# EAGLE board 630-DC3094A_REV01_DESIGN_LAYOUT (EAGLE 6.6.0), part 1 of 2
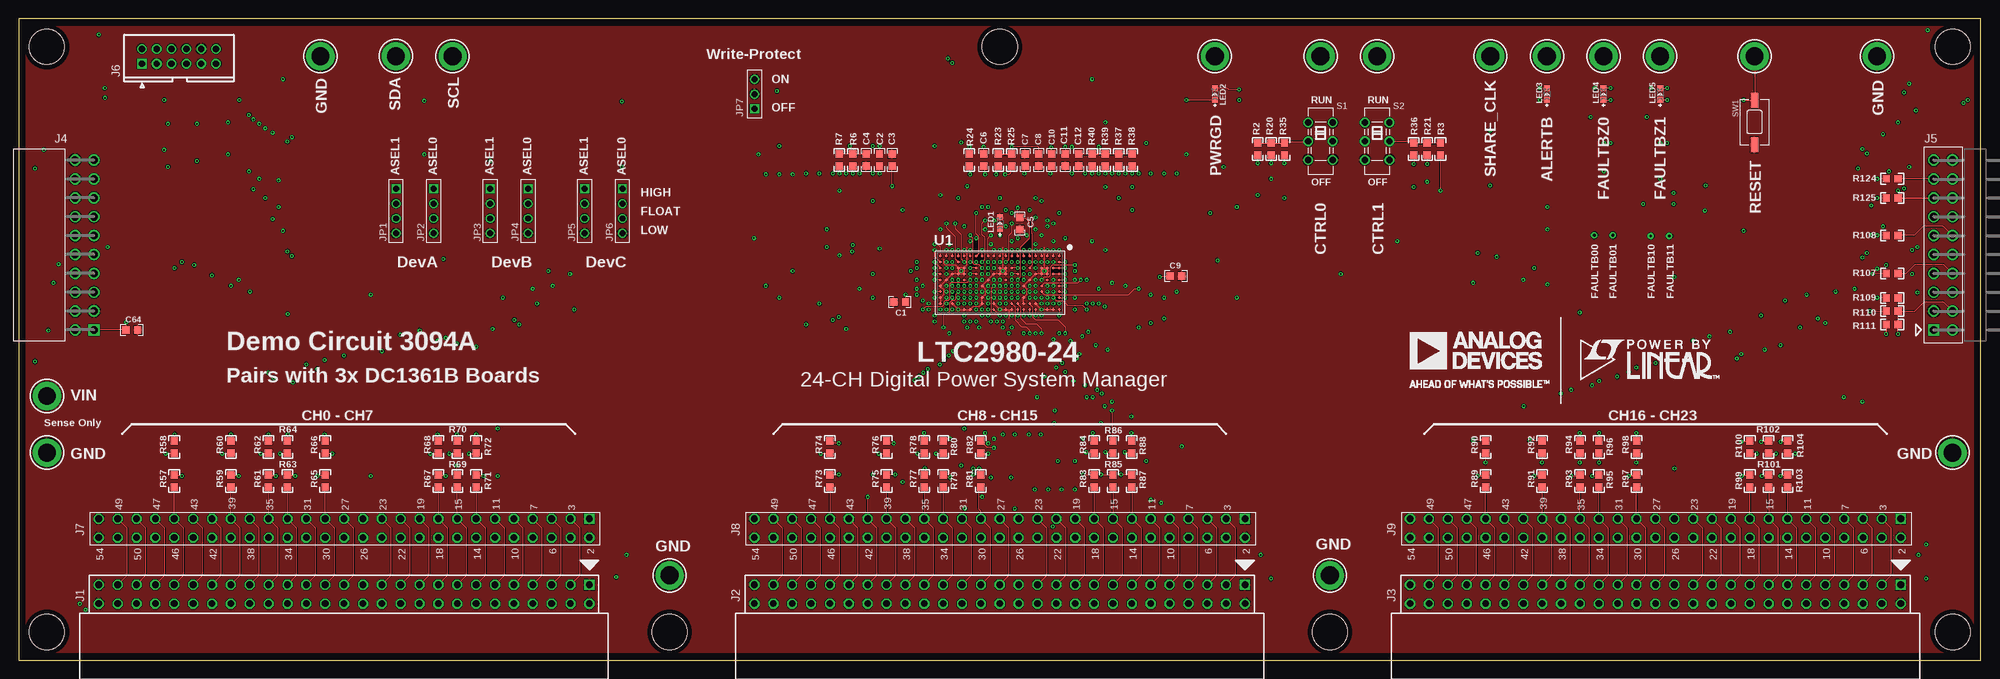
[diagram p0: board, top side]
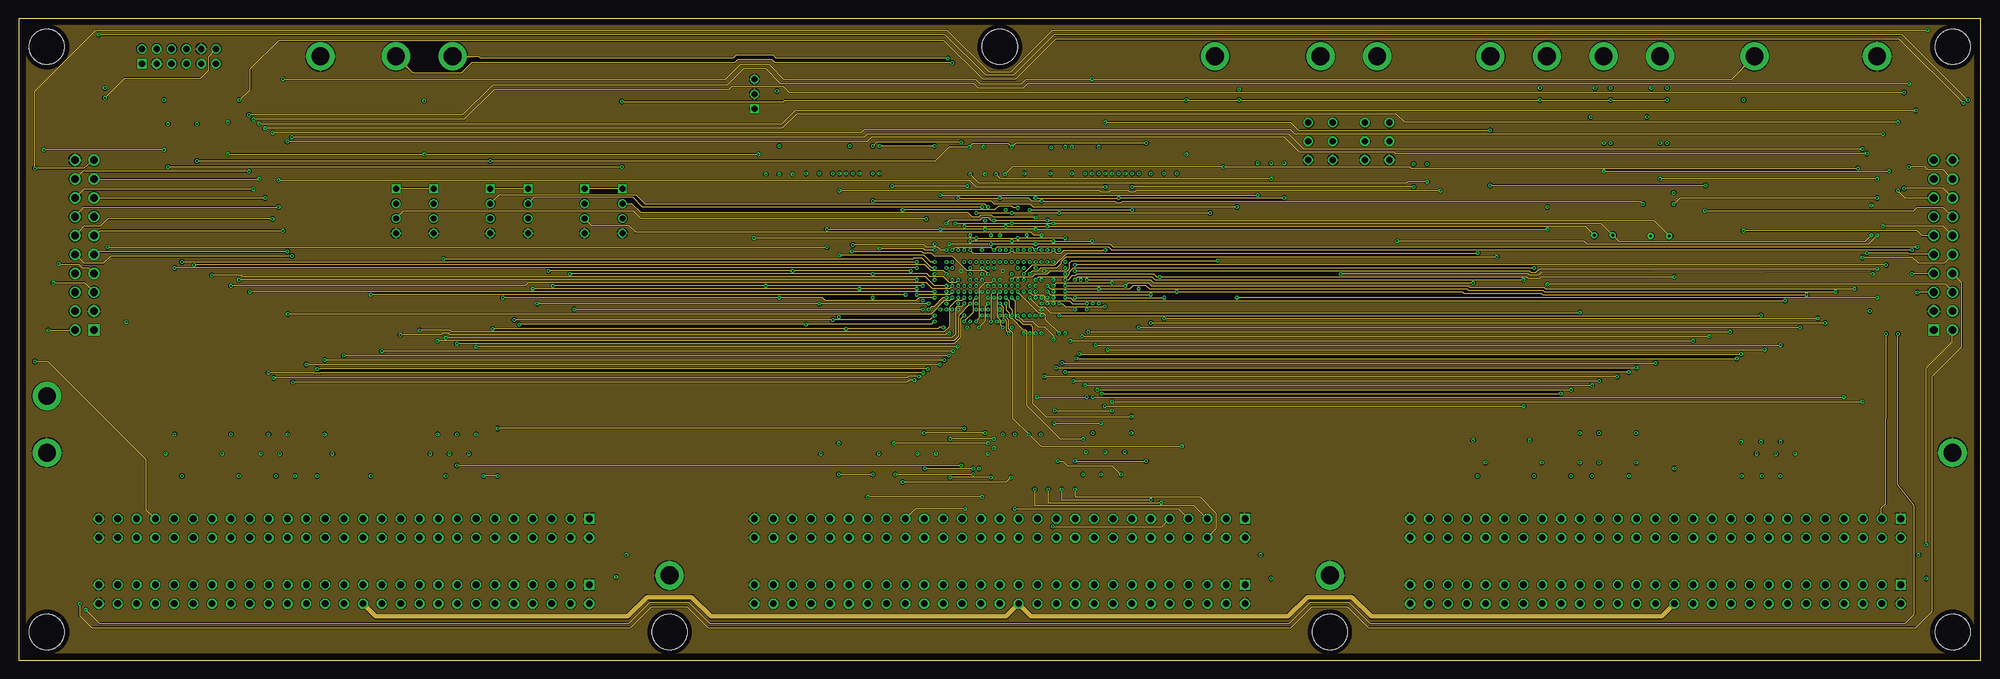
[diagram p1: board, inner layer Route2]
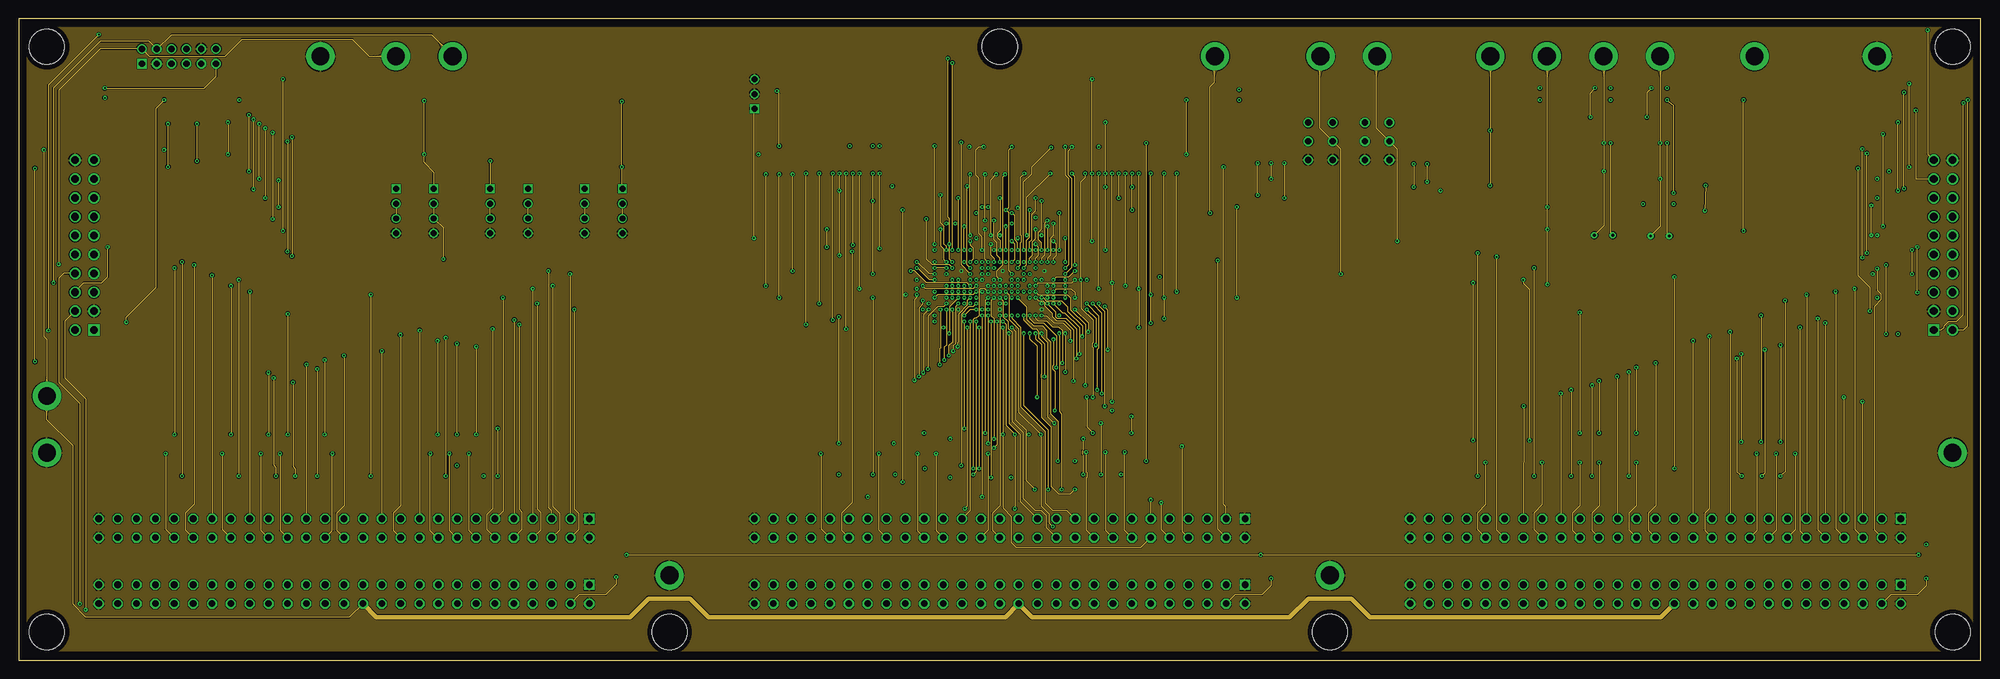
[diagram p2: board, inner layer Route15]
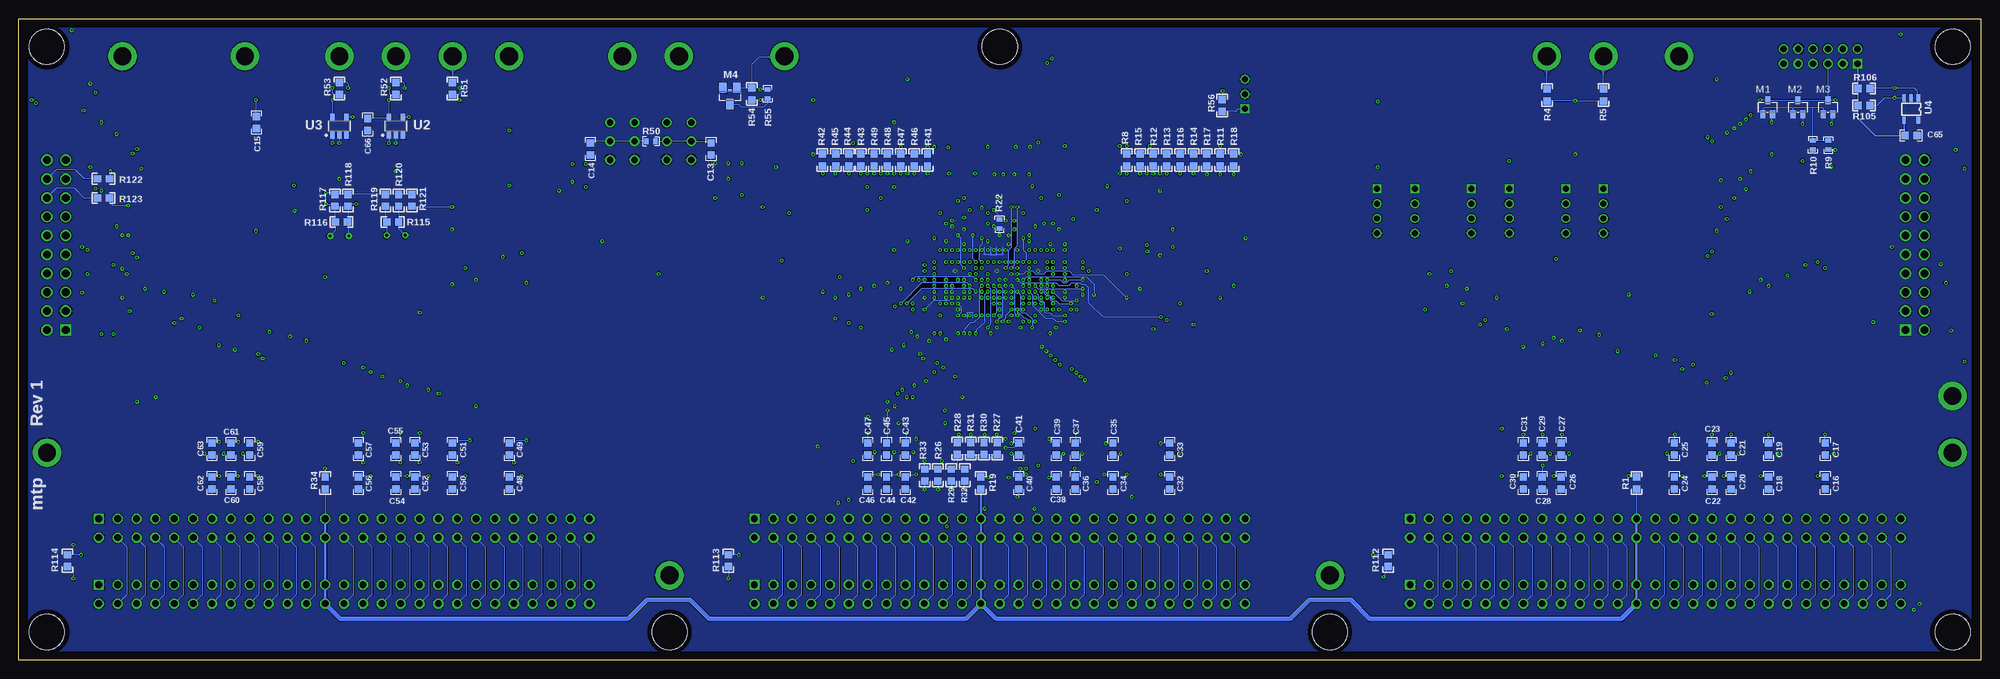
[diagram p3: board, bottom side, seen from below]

Size 264.16 x 86.36 mm. Coordinates in mm from the lower left corner, seen from the top.
Outline: 0,0 264.16,0 264.16,86.36 0,86.36 0,0
Copper layers (1*2+15*16): Top 0.035mm / dielectric 0.25mm / Route2 0.035mm / dielectric 0.9mm / Route15 0.035mm / dielectric 0.25mm / Bottom 0.035mm
Design rules "default *": minimum track width 0.1mm, minimum drill 0.2mm, track to track 0.1mm, track to pad 0.1mm, pad to pad 0.1mm, via to via 0.1mm, smd to smd 0mil, copper to edge 24mil, drill to drill 0.5mm, minimum pad ring 0.15mm, minimum via ring 0.15mm, stop-mask expansion 4mil, vias tented up to drill 10mil, thermal gap 0.15mm
Holes 4.75 mm at 3.81,3.81 3.81,82.55 260.35,82.55 260.35,3.81 87.63,3.81 176.53,3.81 132.08,82.55

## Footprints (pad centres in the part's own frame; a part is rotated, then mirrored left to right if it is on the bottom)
C0603_BOX = smd 1 x 1: 1 -0.8,0; 2 0.8,0
PINHEAD_2X27_RECEPTACLE = drill 0.9 square: 1 1.27,-33.02 | drill 0.9 octagon: 2 -1.27,-33.02; 3 1.27,-30.48; 4 -1.27,-30.48; 5 1.27,-27.94; 6 -1.27,-27.94; 7 1.27,-25.4; 8 -1.27,-25.4; 9 1.27,-22.86; 10 -1.27,-22.86; 11 1.27,-20.32; 12 -1.27,-20.32; 13 1.27,-17.78; 14 -1.27,-17.78; 15 1.27,-15.24; 16 -1.27,-15.24; 17 1.27,-12.7; 18 -1.27,-12.7; 19 1.27,-10.16; 20 -1.27,-10.16; 21 1.27,-7.62; 22 -1.27,-7.62; 23 1.27,-5.08; 24 -1.27,-5.08; 25 1.27,-2.54; 26 -1.27,-2.54; 27 1.27,0; 28 -1.27,0; 29 1.27,2.54; 30 -1.27,2.54; 31 1.27,5.08; 32 -1.27,5.08; 33 1.27,7.62; 34 -1.27,7.62; 35 1.27,10.16; 36 -1.27,10.16; 37 1.27,12.7; 38 -1.27,12.7; 39 1.27,15.24; 40 -1.27,15.24; 41 1.27,17.78; 42 -1.27,17.78; 43 1.27,20.32; 44 -1.27,20.32; 45 1.27,22.86; 46 -1.27,22.86; 47 1.27,25.4; 48 -1.27,25.4; 49 1.27,27.94; 50 -1.27,27.94; 51 1.27,30.48; 52 -1.27,30.48; 53 1.27,33.02; 54 -1.27,33.02
RECEPT_2X10_0.1INCH = drill 1.016 square: P$1 -1.27,11.43 | drill 1.016: P$2 1.27,11.43; P$3 -1.27,8.89; P$4 1.27,8.89; P$5 -1.27,6.35; P$6 1.27,6.35; P$7 -1.27,3.81; P$8 1.27,3.81; P$9 -1.27,1.27; P$10 1.27,1.27; P$11 -1.27,-1.27; P$12 1.27,-1.27; P$13 -1.27,-3.81; P$14 1.27,-3.81; P$15 -1.27,-6.35; P$16 1.27,-6.35; P$17 -1.27,-8.89; P$18 1.27,-8.89; P$19 -1.27,-11.43; P$20 1.27,-11.43
HEADER_2X10_0.1INCH = drill 1.016 square: P$1 1.27,11.43 | drill 1.016: P$2 -1.27,11.43; P$3 1.27,8.89; P$4 -1.27,8.89; P$5 1.27,6.35; P$6 -1.27,6.35; P$7 1.27,3.81; P$8 -1.27,3.81; P$9 1.27,1.27; P$10 -1.27,1.27; P$11 1.27,-1.27; P$12 -1.27,-1.27; P$13 1.27,-3.81; P$14 -1.27,-3.81; P$15 1.27,-6.35; P$16 -1.27,-6.35; P$17 1.27,-8.89; P$18 -1.27,-8.89; P$19 1.27,-11.43; P$20 -1.27,-11.43
CONN_DC1613 = drill 0.86 square: 1 -5,-1 | drill 0.86: 2 -5,1; 3 -3,-1; 4 -3,1; 5 -1,-1; 6 -1,1; 7 1,-1; 8 1,1; 9 3,-1; 10 3,1; 11 5,-1; 12 5,1
PINHEAD_2X27_RECEPTACLE_NO_SILK = drill 0.9 square: 1 1.27,-33.02 | drill 0.9 octagon: 2 -1.27,-33.02; 3 1.27,-30.48; 4 -1.27,-30.48; 5 1.27,-27.94; 6 -1.27,-27.94; 7 1.27,-25.4; 8 -1.27,-25.4; 9 1.27,-22.86; 10 -1.27,-22.86; 11 1.27,-20.32; 12 -1.27,-20.32; 13 1.27,-17.78; 14 -1.27,-17.78; 15 1.27,-15.24; 16 -1.27,-15.24; 17 1.27,-12.7; 18 -1.27,-12.7; 19 1.27,-10.16; 20 -1.27,-10.16; 21 1.27,-7.62; 22 -1.27,-7.62; 23 1.27,-5.08; 24 -1.27,-5.08; 25 1.27,-2.54; 26 -1.27,-2.54; 27 1.27,0; 28 -1.27,0; 29 1.27,2.54; 30 -1.27,2.54; 31 1.27,5.08; 32 -1.27,5.08; 33 1.27,7.62; 34 -1.27,7.62; 35 1.27,10.16; 36 -1.27,10.16; 37 1.27,12.7; 38 -1.27,12.7; 39 1.27,15.24; 40 -1.27,15.24; 41 1.27,17.78; 42 -1.27,17.78; 43 1.27,20.32; 44 -1.27,20.32; 45 1.27,22.86; 46 -1.27,22.86; 47 1.27,25.4; 48 -1.27,25.4; 49 1.27,27.94; 50 -1.27,27.94; 51 1.27,30.48; 52 -1.27,30.48; 53 1.27,33.02; 54 -1.27,33.02
1X04-2MM = drill 0.8 square: 1 -3,0 | drill 0.8: 2 -1,0; 3 1,0; 4 3,0
1X03-2MM = drill 0.8 square: 1 -2,0 | drill 0.8: 2 0,0; 3 2,0
CHIPLED_0603 = smd 0.8 x 0.8: N 0,0.78; P 0,-0.78
SOT323@1 = smd 0.7 x 1.1: 1 -0.65,-0.95; 2 0.65,-0.95; 3 0,0.95
SOT23 = smd 1 x 1.4: 1 -0.95,-1.1; 2 0.95,-1.1; 3 0,1.1
R0603_BOX = smd 1 x 1: 1 -0.8,0; 2 0.8,0
R0402_BOX = smd 0.6 x 0.8: 1 -0.6,0; 2 0.6,0
JS202011CQN = drill 0.86: 1 -2.5,1.65; 2 0,1.65; 3 2.5,1.65; 4 -2.5,-1.65; 5 0,-1.65; 6 2.5,-1.65
SWITCH_PTS635 = smd 2 x 1: SW1 -3,0; SW2 3,0
TURRET_LARGE_2501 = drill 2.388 pad 3.81: TP 0,0
VIA = drill 0.381 pad 0.864: 1 0,0
BGA210 = smd 0.4 x 0.4: A1 -8,-3.6; A2 -8,-2.8; A3 -8,-2; A4 -8,-1.2; A5 -8,-0.4; A6 -8,0.4; A7 -8,1.2; A8 -8,2; A9 -8,2.8; A10 -8,3.6; B1 -7.2,-3.6; B2 -7.2,-2.8; B3 -7.2,-2; B4 -7.2,-1.2; B5 -7.2,-0.4; B6 -7.2,0.4; B7 -7.2,1.2; B8 -7.2,2; B9 -7.2,2.8; B10 -7.2,3.6; C1 -6.4,-3.6; C2 -6.4,-2.8; C3 -6.4,-2; C4 -6.4,-1.2; C5 -6.4,-0.4; C6 -6.4,0.4; C7 -6.4,1.2; C8 -6.4,2; C9 -6.4,2.8; C10 -6.4,3.6; D1 -5.6,-3.6; D2 -5.6,-2.8; D3 -5.6,-2; D4 -5.6,-1.2; D5 -5.6,-0.4; D6 -5.6,0.4; D7 -5.6,1.2; D8 -5.6,2; D9 -5.6,2.8; D10 -5.6,3.6; E1 -4.8,-3.6; E2 -4.8,-2.8; E3 -4.8,-2; E4 -4.8,-1.2; E5 -4.8,-0.4; E6 -4.8,0.4; E7 -4.8,1.2; E8 -4.8,2; E9 -4.8,2.8; E10 -4.8,3.6; F1 -4,-3.6; F2 -4,-2.8; F3 -4,-2; F4 -4,-1.2; F5 -4,-0.4; F6 -4,0.4; F7 -4,1.2; F8 -4,2; F9 -4,2.8; F10 -4,3.6; G1 -3.2,-3.6; G2 -3.2,-2.8; G3 -3.2,-2; G4 -3.2,-1.2; G5 -3.2,-0.4; G6 -3.2,0.4; G7 -3.2,1.2; G8 -3.2,2; G9 -3.2,2.8; G10 -3.2,3.6; H1 -2.4,-3.6; H2 -2.4,-2.8; H3 -2.4,-2; H4 -2.4,-1.2; H5 -2.4,-0.4; H6 -2.4,0.4; H7 -2.4,1.2; H8 -2.4,2; H9 -2.4,2.8; H10 -2.4,3.6; J1 -1.6,-3.6; J2 -1.6,-2.8; J3 -1.6,-2; J4 -1.6,-1.2; J5 -1.6,-0.4; J6 -1.6,0.4; J7 -1.6,1.2; J8 -1.6,2; J9 -1.6,2.8; J10 -1.6,3.6; K1 -0.8,-3.6; K2 -0.8,-2.8; K3 -0.8,-2; K4 -0.8,-1.2; K5 -0.8,-0.4; K6 -0.8,0.4; K7 -0.8,1.2; K8 -0.8,2; K9 -0.8,2.8; K10 -0.8,3.6; L1 0,-3.6; L2 0,-2.8; L3 0,-2; L4 0,-1.2; L5 0,-0.4; L6 0,0.4; L7 0,1.2; L8 0,2; L9 0,2.8; L10 0,3.6; M1 0.8,-3.6; M2 0.8,-2.8; M3 0.8,-2; M4 0.8,-1.2; M5 0.8,-0.4; M6 0.8,0.4; M7 0.8,1.2; M8 0.8,2; M9 0.8,2.8; M10 0.8,3.6; N1 1.6,-3.6; N2 1.6,-2.8; N3 1.6,-2; N4 1.6,-1.2; N5 1.6,-0.4; N6 1.6,0.4; N7 1.6,1.2; N8 1.6,2; N9 1.6,2.8; N10 1.6,3.6; P1 2.4,-3.6; P2 2.4,-2.8; P3 2.4,-2; P4 2.4,-1.2; P5 2.4,-0.4; P6 2.4,0.4; P7 2.4,1.2; P8 2.4,2; P9 2.4,2.8; P10 2.4,3.6; R1 3.2,-3.6; R2 3.2,-2.8; R3 3.2,-2; R4 3.2,-1.2; R5 3.2,-0.4; R6 3.2,0.4; R7 3.2,1.2; R8 3.2,2; R9 3.2,2.8; R10 3.2,3.6; T1 4,-3.6; T2 4,-2.8; T3 4,-2; T4 4,-1.2; T5 4,-0.4; T6 4,0.4; T7 4,1.2; T8 4,2; T9 4,2.8; T10 4,3.6; U1 4.8,-3.6; U2 4.8,-2.8; U3 4.8,-2; U4 4.8,-1.2; U5 4.8,-0.4; U6 4.8,0.4; U7 4.8,1.2; U8 4.8,2; U9 4.8,2.8; U10 4.8,3.6; W1 5.6,-3.6; W2 5.6,-2.8; W3 5.6,-2; W4 5.6,-1.2; W5 5.6,-0.4; W6 5.6,0.4; W7 5.6,1.2; W8 5.6,2; W9 5.6,2.8; W10 5.6,3.6; X1 6.4,-3.6; X2 6.4,-2.8; X3 6.4,-2; X4 6.4,-1.2; X5 6.4,-0.4; X6 6.4,0.4; X7 6.4,1.2; X8 6.4,2; X9 6.4,2.8; X10 6.4,3.6; Y1 7.2,-3.6; Y2 7.2,-2.8; Y3 7.2,-2; Y4 7.2,-1.2; Y5 7.2,-0.4; Y6 7.2,0.4; Y7 7.2,1.2; Y8 7.2,2; Y9 7.2,2.8; Y10 7.2,3.6; Z1 8,-3.6; Z2 8,-2.8; Z3 8,-2; Z4 8,-1.2; Z5 8,-0.4; Z6 8,0.4; Z7 8,1.2; Z8 8,2; Z9 8,2.8; Z10 8,3.6
SOT23-5 = smd 0.6 x 1: 1 -0.95,-1.2; 2 0,-1.2; 3 0.95,-1.2; 4 0.95,1.2; 5 -0.95,1.2
SOT-23-5 = smd 1 x 0.5: 1 -1.491,0.95; 2 -1.491,0; 3 -1.491,-0.95; 4 1.491,-0.95; 5 1.491,0.95

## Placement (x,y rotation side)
C1  0.1uF  [C0603_BOX]  118.6,48.2 180 top
C2  0.1uF  [C0603_BOX]  115.9,67.31 90 top
C3  0.1uF  [C0603_BOX]  117.6,67.31 90 top
C4  0.1uF  [C0603_BOX]  114.1,67.31 270 top
C5  0.1uF  [C0603_BOX]  134.8,58.8 270 top
C6  0.1uF  [C0603_BOX]  129.9,67.31 90 top
C7  0.1uF  [C0603_BOX]  135.5,67.31 90 top
C8  0.1uF  [C0603_BOX]  137.3,67.31 270 top
C9  0.1uF  [C0603_BOX]  155.8,51.7 0 top
C10  0.1uF  [C0603_BOX]  139.09,67.31 90 top
C11  0.1uF  [C0603_BOX]  140.9,67.31 270 top
C12  0.1uF  [C0603_BOX]  142.7,67.31 270 top
C13  1uF  [C0603_BOX]  170.94,68.8 270 bottom
C14  1uF  [C0603_BOX]  187.2,68.8 270 bottom
C15  10n  [C0603_BOX]  232.16,72.39 90 bottom
C16  100n  [C0603_BOX]  20.95,23.88 270 bottom
C17  100n  [C0603_BOX]  20.95,28.45 270 bottom
C18  100n  [C0603_BOX]  28.57,23.88 270 bottom
C19  100n  [C0603_BOX]  28.57,28.45 270 bottom
C20  100n  [C0603_BOX]  33.66,23.88 270 bottom
C21  100n  [C0603_BOX]  33.66,28.45 270 bottom
C22  100n  [C0603_BOX]  36.2,23.88 270 bottom
C23  100n  [C0603_BOX]  36.2,28.45 270 bottom
C24  100n  [C0603_BOX]  41.27,23.88 270 bottom
C25  100n  [C0603_BOX]  41.27,28.45 270 bottom
C26  100n  [C0603_BOX]  56.52,23.88 270 bottom
C27  100n  [C0603_BOX]  56.52,28.45 270 bottom
C28  100n  [C0603_BOX]  59.05,23.88 270 bottom
C29  100n  [C0603_BOX]  59.05,28.45 270 bottom
C30  100n  [C0603_BOX]  61.59,23.88 270 bottom
C31  100n  [C0603_BOX]  61.59,28.45 270 bottom
C32  100n  [C0603_BOX]  109.22,23.88 270 bottom
C33  100n  [C0603_BOX]  109.22,28.45 270 bottom
C34  100n  [C0603_BOX]  116.84,23.88 270 bottom
C35  100n  [C0603_BOX]  116.84,28.45 270 bottom
C36  100n  [C0603_BOX]  121.92,23.88 270 bottom
C37  100n  [C0603_BOX]  121.92,28.45 270 bottom
C38  100n  [C0603_BOX]  124.46,23.88 270 bottom
C39  100n  [C0603_BOX]  124.46,28.45 270 bottom
C40  100n  [C0603_BOX]  129.5,23.88 270 bottom
C41  100n  [C0603_BOX]  129.54,28.45 270 bottom
C42  100n  [C0603_BOX]  144.78,23.88 270 bottom
C43  100n  [C0603_BOX]  144.78,28.45 270 bottom
C44  100n  [C0603_BOX]  147.32,23.88 270 bottom
C45  100n  [C0603_BOX]  147.32,28.45 270 bottom
C46  100n  [C0603_BOX]  149.86,23.88 270 bottom
C47  100n  [C0603_BOX]  149.86,28.45 270 bottom
C48  100n  [C0603_BOX]  198.12,23.88 270 bottom
C49  100n  [C0603_BOX]  198.12,28.45 270 bottom
C50  100n  [C0603_BOX]  205.74,23.88 270 bottom
C51  100n  [C0603_BOX]  205.74,28.45 270 bottom
C52  100n  [C0603_BOX]  210.82,23.88 270 bottom
C53  100n  [C0603_BOX]  210.82,28.45 270 bottom
C54  100n  [C0603_BOX]  213.36,23.88 270 bottom
C55  100n  [C0603_BOX]  213.36,28.45 270 bottom
C56  100n  [C0603_BOX]  218.44,23.88 270 bottom
C57  100n  [C0603_BOX]  218.44,28.45 270 bottom
C58  100n  [C0603_BOX]  233.04,23.88 270 bottom
C59  100n  [C0603_BOX]  233.04,28.45 270 bottom
C60  100n  [C0603_BOX]  235.59,23.88 270 bottom
C61  100n  [C0603_BOX]  235.59,28.45 270 bottom
C62  100n  [C0603_BOX]  238.12,23.88 270 bottom
C63  100n  [C0603_BOX]  238.12,28.45 270 bottom
C64  1uF  [C0603_BOX]  15.24,44.45 0 top
C65  1uF  [C0603_BOX]  9.4,70.61 0 bottom
C66  0.1uF  [C0603_BOX]  217.17,72.1 270 bottom
DRILEGEND  [DRILEGEND]  not placed on the board
J1  CONN_2X27F  [PINHEAD_2X27_RECEPTACLE]  43.81,8.89 90 top
J2  CONN_2X27F  [PINHEAD_2X27_RECEPTACLE]  132.08,8.89 90 top
J3  CONN_2X27F  [PINHEAD_2X27_RECEPTACLE]  220.34,8.89 90 top
J4  RECEPT_CONN_2X10_0.1INCH  [RECEPT_2X10_0.1INCH]  8.89,55.88 180 top
J5  HEADER_CONN_2X10_0.1INCH  [HEADER_2X10_0.1INCH]  259.08,55.88 180 top
J6  CONN_DC1613  [CONN_DC1613]  21.59,81.28 0 top
J7  CONN_2X27_NO_SILK  [PINHEAD_2X27_RECEPTACLE_NO_SILK]  43.81,17.78 90 top
J8  CONN_2X27_NO_SILK  [PINHEAD_2X27_RECEPTACLE_NO_SILK]  132.08,17.78 90 top
J9  CONN_2X27_NO_SILK  [PINHEAD_2X27_RECEPTACLE_NO_SILK]  220.34,17.78 90 top
JP1  [1X04-2MM]  50.8,60.45 270 top
JP2  [1X04-2MM]  55.88,60.45 270 top
JP3  [1X04-2MM]  63.5,60.45 270 top
JP4  [1X04-2MM]  68.58,60.45 270 top
JP5  [1X04-2MM]  76.2,60.45 270 top
JP6  [1X04-2MM]  81.28,60.45 270 top
JP7  [1X03-2MM]  99.06,76.2 90 top
LED1  GREEN  [CHIPLED_0603]  132.1,58.83 0 top
LED2  GREEN  [CHIPLED_0603]  161.04,76.2 0 top
LED3  RED  [CHIPLED_0603]  205.74,76.2 0 top
LED4  RED  [CHIPLED_0603]  213.36,76.2 0 top
LED5  RED  [CHIPLED_0603]  220.98,76.2 0 top
M1  NTS4173P  [SOT323@1]  28.7,74.42 0 bottom
M2  NTS4173P  [SOT323@1]  24.64,74.42 0 bottom
M3  NTS4173P  [SOT323@1]  20.57,74.42 0 bottom
M4  2N7002  [SOT23]  168.4,75.95 180 bottom
R1  10  [R0603_BOX]  46.35,23.88 90 bottom
R2  0  [R0603_BOX]  166.8,68.8 270 top
R3  0  [R0603_BOX]  191.4,68.8 270 top
R4  10k  [R0603_BOX]  58.42,76.09 90 bottom
R5  10k  [R0603_BOX]  50.8,76.09 90 bottom
R6  20k  [R0603_BOX]  112.3,67.31 90 top
R7  20k  [R0603_BOX]  110.5,67.31 90 top
R8  20k  [R0603_BOX]  115,67.31 90 bottom
R9  49.9k  [R0402_BOX]  20.57,69.34 90 bottom
R10  150k  [R0402_BOX]  22.61,69.34 270 bottom
R11  10k  [R0603_BOX]  102.4,67.31 90 bottom
R12  10k  [R0603_BOX]  111.4,67.31 90 bottom
R13  10k  [R0603_BOX]  109.6,67.31 90 bottom
R14  10k  [R0603_BOX]  106,67.31 90 bottom
R15  10k  [R0603_BOX]  113.2,67.31 90 bottom
R16  10k  [R0603_BOX]  107.8,67.31 90 bottom
R17  10k  [R0603_BOX]  104.2,67.31 90 bottom
R18  10k  [R0603_BOX]  100.6,67.31 90 bottom
R19  10  [R0603_BOX]  134.62,23.88 90 bottom
R20  0  [R0603_BOX]  168.6,68.8 270 top
R21  0  [R0603_BOX]  189.6,68.8 270 top
R22  15k  [R0402_BOX]  132.1,58.7 90 bottom
R23  20k  [R0603_BOX]  131.9,67.31 90 top
R24  20k  [R0603_BOX]  128,67.31 90 top
R25  20k  [R0603_BOX]  133.7,67.31 90 top
R26  10k  [R0603_BOX]  140.4,24.91 90 bottom
R27  10k  [R0603_BOX]  132.4,28.49 270 bottom
R28  10k  [R0603_BOX]  137.8,28.49 270 bottom
R29  10k  [R0603_BOX]  138.6,24.91 90 bottom
R30  10k  [R0603_BOX]  134.2,28.49 270 bottom
R31  10k  [R0603_BOX]  136,28.49 270 bottom
R32  10k  [R0603_BOX]  136.8,24.91 90 bottom
R33  10k  [R0603_BOX]  142.2,24.91 90 bottom
R34  10  [R0603_BOX]  222.88,23.88 90 bottom
R35  0  [R0603_BOX]  170.4,68.8 270 top
R36  0  [R0603_BOX]  187.8,68.8 270 top
R37  20k  [R0603_BOX]  148.1,67.31 90 top
R38  20k  [R0603_BOX]  149.9,67.31 90 top
R39  5.49k  [R0603_BOX]  146.3,67.31 90 top
R40  10k  [R0603_BOX]  144.5,67.31 90 top
R41  20k  [R0603_BOX]  141.8,67.31 90 bottom
R42  10k  [R0603_BOX]  155.96,67.31 90 bottom
R43  10k  [R0603_BOX]  150.8,67.31 90 bottom
R44  10k  [R0603_BOX]  152.4,67.31 90 bottom
R45  10k  [R0603_BOX]  154.18,67.31 90 bottom
R46  10k  [R0603_BOX]  143.6,67.31 90 bottom
R47  10k  [R0603_BOX]  145.4,67.31 90 bottom
R48  10k  [R0603_BOX]  147.2,67.31 90 bottom
R49  10k  [R0603_BOX]  149,67.31 90 bottom
R50  0  [R0402_BOX]  179.07,69.85 0 bottom
R51  499  [R0603_BOX]  205.74,76.96 270 bottom
R52  499  [R0603_BOX]  213.36,76.96 90 bottom
R53  499  [R0603_BOX]  220.98,76.96 90 bottom
R54  10k  [R0603_BOX]  165.45,76.2 270 bottom
R55  15k  [R0402_BOX]  163.32,76.2 270 bottom
R56  10k  [R0603_BOX]  102.11,74.68 90 bottom
R57  100  [R0603_BOX]  20.95,24.13 90 top
R58  100  [R0603_BOX]  20.95,28.7 90 top
R59  100  [R0603_BOX]  28.57,24.13 90 top
R60  100  [R0603_BOX]  28.57,28.7 90 top
R61  100  [R0603_BOX]  33.66,24.13 90 top
R62  100  [R0603_BOX]  33.66,28.7 90 top
R63  100  [R0603_BOX]  36.2,24.13 90 top
R64  100  [R0603_BOX]  36.2,28.7 90 top
R65  100  [R0603_BOX]  41.27,24.13 90 top
R66  100  [R0603_BOX]  41.27,28.7 90 top
R67  100  [R0603_BOX]  56.52,24.13 90 top
R68  100  [R0603_BOX]  56.52,28.7 90 top
R69  100  [R0603_BOX]  59.05,24.13 90 top
R70  100  [R0603_BOX]  59.05,28.7 90 top
R71  100  [R0603_BOX]  61.59,24.13 90 top
R72  100  [R0603_BOX]  61.59,28.7 90 top
R73  100  [R0603_BOX]  109.22,24.13 90 top
R74  100  [R0603_BOX]  109.22,28.7 90 top
R75  100  [R0603_BOX]  116.84,24.13 90 top
R76  100  [R0603_BOX]  116.84,28.7 90 top
R77  100  [R0603_BOX]  121.92,24.13 90 top
R78  100  [R0603_BOX]  121.92,28.7 90 top
R79  100  [R0603_BOX]  124.46,24.13 90 top
R80  100  [R0603_BOX]  124.46,28.7 90 top
R81  100  [R0603_BOX]  129.5,24.13 90 top
R82  100  [R0603_BOX]  129.54,28.7 90 top
R83  100  [R0603_BOX]  144.78,24.13 90 top
R84  100  [R0603_BOX]  144.78,28.7 90 top
R85  100  [R0603_BOX]  147.32,24.13 90 top
R86  100  [R0603_BOX]  147.32,28.7 90 top
R87  100  [R0603_BOX]  149.86,24.13 90 top
R88  100  [R0603_BOX]  149.86,28.7 90 top
R89  100  [R0603_BOX]  197.49,24.13 90 top
R90  100  [R0603_BOX]  197.49,28.7 90 top
R91  100  [R0603_BOX]  205.1,24.13 90 top
R92  100  [R0603_BOX]  205.1,28.7 90 top
R93  100  [R0603_BOX]  210.19,24.13 90 top
R94  100  [R0603_BOX]  210.19,28.7 90 top
R95  100  [R0603_BOX]  212.72,24.13 90 top
R96  100  [R0603_BOX]  212.72,28.7 90 top
R97  100  [R0603_BOX]  217.81,24.13 90 top
R98  100  [R0603_BOX]  217.81,28.7 90 top
R99  100  [R0603_BOX]  233.04,24.13 90 top
R100  100  [R0603_BOX]  233.04,28.7 90 top
R101  100  [R0603_BOX]  235.59,24.13 90 top
R102  100  [R0603_BOX]  235.59,28.7 90 top
R103  100  [R0603_BOX]  238.12,24.13 90 top
R104  100  [R0603_BOX]  238.12,28.7 90 top
R105  10k  [R0603_BOX]  15.75,74.68 180 bottom
R106  10k  [R0603_BOX]  15.75,76.96 180 bottom
R107  1k  [R0603_BOX]  252.22,52.07 0 top
R108  1k  [R0603_BOX]  252.22,57.15 0 top
R109  0 (DNI)  [R0603_BOX]  252.22,48.77 180 top
R110  0 (DNI)  [R0603_BOX]  252.22,46.99 180 top
R111  0 (DNI)  [R0603_BOX]  252.22,45.21 180 top
R112  0 (DNI)  [R0603_BOX]  79.8,13.4 270 bottom
R113  0 (DNI)  [R0603_BOX]  168.6,13.4 270 bottom
R114  0 (DNI)  [R0603_BOX]  257.6,13.4 270 bottom
R115  0 (DNI)  [R0603_BOX]  213.8,59 0 bottom
R116  0 (DNI)  [R0603_BOX]  220.7,59 0 bottom
R117  20k  [R0603_BOX]  221.6,61.9 90 bottom
R118  20k  [R0603_BOX]  219.8,61.9 90 bottom
R119  20k  [R0603_BOX]  214.8,61.9 90 bottom
R120  20k  [R0603_BOX]  213,61.9 90 bottom
R121  10k  [R0603_BOX]  211.2,61.9 90 bottom
R122  0  [R0603_BOX]  252.73,64.8 0 bottom
R123  0  [R0603_BOX]  252.73,62.2 0 bottom
R124  0  [R0603_BOX]  252.22,64.8 180 top
R125  0  [R0603_BOX]  252.22,62.2 180 top
S1  CONTROL0  [JS202011CQN]  175.26,69.85 270 top
S2  CONTROL1  [JS202011CQN]  182.88,69.85 270 top
SW1  PTS635SL25SMTR LFS  [SWITCH_PTS635]  233.68,72.39 270 top
TP1  [TURRET_LARGE_2501]  58.42,81.28 0 top
TP2  [TURRET_LARGE_2501]  50.8,81.3 0 top
TP3  [TURRET_LARGE_2501]  205.74,81.28 0 top
TP4  [TURRET_LARGE_2501]  213.36,81.28 0 top
TP5  [TURRET_LARGE_2501]  220.98,81.28 0 top
TP6  [TURRET_LARGE_2501]  198.12,81.28 0 top
TP7  [TURRET_LARGE_2501]  233.68,81.28 0 top
TP8  [TURRET_LARGE_2501]  161.04,81.28 0 top
TP9  [TURRET_LARGE_2501]  3.81,35.56 0 top
TP10  TESTPOINTVIA  [VIA]  212.1,57.2 90 top
TP11  TESTPOINTVIA  [VIA]  214.6,57.2 90 top
TP12  TESTPOINTVIA  [VIA]  219.7,57.1 90 top
TP13  TESTPOINTVIA  [VIA]  222.2,57.1 90 top
TP14  [TURRET_LARGE_2501]  175.26,81.28 0 top
TP15  [TURRET_LARGE_2501]  182.88,81.28 0 top
TP16  [TURRET_LARGE_2501]  3.81,27.94 90 top
TP17  [TURRET_LARGE_2501]  260.35,27.94 90 top
TP18  [TURRET_LARGE_2501]  40.64,81.28 90 top
TP19  [TURRET_LARGE_2501]  250.19,81.28 90 top
TP20  [TURRET_LARGE_2501]  87.63,11.43 0 top
TP21  [TURRET_LARGE_2501]  176.53,11.43 0 top
U1  LTC2980-24  [BGA210]  132.1,50.8 180 top
U2  74*1G09  [SOT23-5]  213.36,71.88 0 bottom
U3  74*1G09  [SOT23-5]  220.98,71.88 0 bottom
U4  24AA02T-I/OT  [SOT-23-5]  9.4,74.17 270 bottom
U$2  [DC3094_FRAME]  not placed on the board
U$110  [LOGO-ADI-POWER-BY-LINEAR-1650MILS-POS-SILK]  187.09,34.35 0 top

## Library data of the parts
C1-C66 = rcl
DRILEGEND = drilegend
J1-J3 J7-J9 JP1-JP7 = pinhead
J4 J5 = con-millmax
J6 = con-fci
LED1-LED5 = led
M1-M4 = transistor-fet
R1-R125 = resistor
S1 S2 SW1 U4 = kalin
TP1-TP21 = testpad
U1 U$110 = linear-technology
U2 U3 = 74xx-little-us
U$2 = frames

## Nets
ALERTB: J4.P$6 J5.P$6 R51.1 R121.1 TP3.TP U1.F2 U1.N2 U1.Y2
ASEL0_A: JP2.2 JP2.3 U1.Y3
ASEL0_B: JP4.2 JP4.3 U1.N3
ASEL0_C: JP6.2 JP6.3 U1.F3
ASEL1_A: JP1.2 JP1.3 U1.X3
ASEL1_B: JP3.2 JP3.3 U1.M3
ASEL1_C: JP5.2 JP5.3 U1.E3
AUX_SCL: J6.11 R106.1 U4.1
AUX_SDA: J6.12 R105.1 U4.3
AUXFAULTB_3V3: J4.P$4 J5.P$4 R109.1 R110.1 R111.1
CTRL0: C13.1 R2.1 R20.1 R35.1 R50.2 R107.1 S1.2 S1.5 TP14.TP
CTRL0_A: R35.2 R37.1 U1.F1
CTRL0_B: R20.2 R23.1 U1.N1
CTRL0_C: R2.2 R6.1 U1.Y1
CTRL0_X: J4.P$8 J5.P$8 R107.2
CTRL1: C14.1 R3.1 R21.1 R36.1 R50.1 R108.1 S2.2 S2.5 TP15.TP
CTRL1_A: R36.2 R38.1 U1.G3
CTRL1_B: R21.2 R24.1 U1.P3
CTRL1_C: R3.2 R7.1 U1.Z3
CTRL1_X: J4.P$12 J5.P$12 R108.2
CTRL2: J4.P$9 J5.P$9
CTRL3: J4.P$10 J5.P$10
DACM_CH0: J1.43 J7.43
DACM_CH1: J1.42 J7.42
DACM_CH2: J1.38 J7.38
DACM_CH3: J1.32 J7.32
DACM_CH4: J1.27 J7.27
DACM_CH5: J1.24 J7.24
DACM_CH6: J1.21 J7.21
DACM_CH7: J1.20 J7.20
DACM_CH8: J2.43 J8.43
DACM_CH9: J2.42 J8.42
DACM_CH10: J2.38 J8.38
DACM_CH11: J2.32 J8.32
DACM_CH12: J2.27 J8.27
DACM_CH13: J2.24 J8.24
DACM_CH14: J2.21 J8.21
DACM_CH15: J2.20 J8.20
DACM_CH16: J3.43 J9.43
DACM_CH17: J3.42 J9.42
DACM_CH18: J3.38 J9.38
DACM_CH19: J3.32 J9.32
DACM_CH20: J3.27 J9.27
DACM_CH21: J3.24 J9.24
DACM_CH22: J3.21 J9.21
DACM_CH23: J3.20 J9.20
DACP_CH0: J1.44 J7.44 U1.Y4
DACP_CH1: J1.41 J7.41 U1.Y6
DACP_CH2: J1.37 J7.37 U1.Z7
DACP_CH3: J1.31 J7.31 U1.Z10
DACP_CH4: J1.28 J7.28 U1.X10
DACP_CH5: J1.23 J7.23 U1.W9
DACP_CH6: J1.22 J7.22 U1.W8
DACP_CH7: J1.19 J7.19 U1.U8
DACP_CH8: J2.44 J8.44 U1.N4
DACP_CH9: J2.41 J8.41 U1.N6
DACP_CH10: J2.37 J8.37 U1.P7
DACP_CH11: J2.31 J8.31 U1.P10
DACP_CH12: J2.28 J8.28 U1.M10
DACP_CH13: J2.23 J8.23 U1.L9
DACP_CH14: J2.22 J8.22 U1.L8
DACP_CH15: J2.19 J8.19 U1.K8
DACP_CH16: J3.44 J9.44 U1.F4
DACP_CH17: J3.41 J9.41 U1.F6
DACP_CH18: J3.37 J9.37 U1.G7
DACP_CH19: J3.31 J9.31 U1.G10
DACP_CH20: J3.28 J9.28 U1.E10
DACP_CH21: J3.23 J9.23 U1.D9
DACP_CH22: J3.22 J9.22 U1.D8
DACP_CH23: J3.19 J9.19 U1.C8
FAULT1: J4.P$18 J5.P$18 R122.1
FAULT2: J4.P$16 J5.P$16 R123.1
FAULT3: J4.P$17 J5.P$17 R124.1
FAULT4: J4.P$15 J5.P$15 R125.1
FAULTB00: R115.2 R120.1 R122.2 TP4.TP TP10.1 U1.C1 U1.K1 U1.U1 U2.2
FAULTB01: R115.1 R119.1 R123.2 TP11.1 U1.C2 U1.K2 U1.U2 U2.1
FAULTB10: R116.2 R118.1 R124.2 TP5.TP TP12.1 U1.D1 U1.L1 U1.W1 U3.2
FAULTB11: R116.1 R117.1 R125.2 TP13.1 U1.D2 U1.L2 U1.W2 U3.1
FAULTBZ0: R52.2 U2.4
FAULTBZ1: R53.2 U3.4
GND: C1.2 C3.2 C4.2 C5.2 C7.2 C8.2 C9.2 C11.2 C12.2 C13.2 C14.2 C15.1 C16.2 C17.2 C18.2 C19.2 C20.2 C21.2 C22.2 C23.2 C24.2 C25.2 C26.2 C27.2 C28.2 C29.2 C30.2 C31.2 C32.2 C33.2 C34.2 C35.2 C36.2 C37.2 C38.2 C39.2 C40.2 C41.2 C42.2 C43.2 C44.2 C45.2 C46.2 C47.2 C48.2 C49.2 C50.2 C51.2 C52.2 C53.2 C54.2 C55.2 C56.2 C57.2 C58.2 C59.2 C60.2 C61.2 C62.2 C63.2 C64.2 C65.2 C66.2 J1.1 J1.2 J1.53 J1.54 J2.1 J2.2 J2.53 J2.54 J3.1 J3.2 J3.53 J3.54 J4.P$3 J4.P$20 J5.P$3 J5.P$20 J6.3 J6.10 J7.1 J7.2 J7.53 J7.54 J8.1 J8.2 J8.53 J8.54 J9.1 J9.2 J9.53 J9.54 JP1.4 JP2.4 JP3.4 JP4.4 JP5.4 JP6.4 JP7.2 JP7.3 LED1.N M4.2 R10.2 S1.3 S1.6 S2.3 S2.6 SW1.SW2 TP16.TP TP17.TP TP18.TP TP19.TP TP20.TP TP21.TP U1.B10 U1.C3 U1.C4 U1.C10 U1.D3 U1.D4 U1.D10 U1.E4 U1.E9 U1.F5 U1.G6 U1.G8 U1.G9 U1.J10 U1.K3 U1.K4 U1.K10 U1.L3 U1.L4 U1.L10 U1.M4 U1.M9 U1.N5 U1.P6 U1.P8 U1.P9 U1.T10 U1.U3 U1.U4 U1.U10 U1.W3 U1.W4 U1.W10 U1.X4 U1.X9 U1.Y5 U1.Z6 U1.Z8 U1.Z9 U2.3 U3.3 U4.2 U4.5
N$2: LED2.N R55.1
N$4: LED1.P R22.1
N$8: M4.3 R55.2
N$16: J4.P$13
N$28: LED5.N R53.1
N$29: LED4.N R52.1
N$30: LED3.N R51.2
PFET_GATE: M1.1 M2.1 M3.1 R9.2 R10.1
PGOOD3: J5.P$13
PWRGD: M4.1 R54.1 TP8.TP U1.A1 U1.H1 U1.R1
PWRGD_A: J1.49 J7.49
PWRGD_B: J2.49 J8.49
PWRGD_C: J3.49 J9.49
REFM_A: C10.2 U1.G1
REFM_B: C6.2 U1.P1
REFM_C: C2.2 U1.Z1
REFP_A: C10.1 U1.G2
REFP_B: C6.1 U1.P2
REFP_C: C2.1 U1.Z2
RESETB: C15.2 J4.P$11 J5.P$11 R40.1 SW1.SW1 TP7.TP U1.B2 U1.J2 U1.T2
RUN_CH0: J1.11 J7.11 R11.1 U1.R7
RUN_CH1: J1.12 J7.12 R12.1 U1.W7
RUN_CH2: J1.9 J7.9 R13.1 U1.U7
RUN_CH3: J1.10 J7.10 R14.1 U1.T7
RUN_CH4: J1.7 J7.7 R15.1 U1.W6
RUN_CH5: J1.8 J7.8 R16.1 U1.U6
RUN_CH6: J1.5 J7.5 R17.1 U1.T6
RUN_CH7: J1.6 J7.6 R18.1 U1.R6
RUN_CH8: J2.11 J8.11 R26.1 U1.H7
RUN_CH9: J2.12 J8.12 R27.1 U1.L7
RUN_CH10: J2.9 J8.9 R28.1 U1.K7
RUN_CH11: J2.10 J8.10 R29.1 U1.J7
RUN_CH12: J2.7 J8.7 R30.1 U1.L6
RUN_CH13: J2.8 J8.8 R31.1 U1.K6
RUN_CH14: J2.5 J8.5 R32.1 U1.J6
RUN_CH15: J2.6 J8.6 R33.1 U1.H6
RUN_CH16: J3.11 J9.11 R42.1 U1.A7
RUN_CH17: J3.12 J9.12 R43.1 U1.D7
RUN_CH18: J3.9 J9.9 R44.1 U1.C7
RUN_CH19: J3.10 J9.10 R45.1 U1.B7
RUN_CH20: J3.7 J9.7 R46.1 U1.D6
RUN_CH21: J3.8 J9.8 R47.1 U1.C6
RUN_CH22: J3.5 J9.5 R48.1 U1.B6
RUN_CH23: J3.6 J9.6 R49.1 U1.A6
SCL: J4.P$5 J5.P$5 J6.4 R4.2 TP1.TP U1.E2 U1.M2 U1.X2
SDA: J4.P$7 J5.P$7 J6.2 R5.2 TP2.TP U1.E1 U1.M1 U1.X1
SHARE_CLK: J4.P$14 J5.P$14 R39.1 TP6.TP U1.B1 U1.J1 U1.T1
SPARE1: J1.48 J7.48
SPARE2: J1.50 J7.50
SPARE3: J1.52 J7.52
SPARE4: J1.47 J4.P$19 J5.P$19 J7.47
SPARE5: J1.51 J7.51
SPARE6: J2.48 J8.48
SPARE7: J2.50 J8.50
SPARE8: J2.52 J8.52
SPARE9: J2.47 J8.47
SPARE10: J2.51 J8.51
SPARE11: J3.48 J9.48
SPARE12: J3.50 J9.50
SPARE13: J3.52 J9.52
SPARE14: J3.47 J9.47
SPARE15: J3.51 J9.51
USB_3.3V: C64.1 J4.P$1 J5.P$1 J6.5 M1.3 M2.3 M3.3
USB_5V: C65.1 J6.1 R105.2 R106.2 U4.4
VDD25_A: C11.1 U1.A3 U1.B3
VDD25_B: C7.1 U1.H3 U1.J3
VDD25_C: C3.1 U1.R3 U1.T3
VDD33_A: C4.1 JP1.1 JP2.1 M1.2 R4.1 R5.1 R6.2 R7.2 R8.2 R11.2 R12.2 R13.2 R14.2 R15.2 R16.2 R17.2 R18.2 R56.2 U1.R4 U1.T4
VDD33_B: C8.1 JP3.1 JP4.1 M2.2 R22.2 R23.2 R24.2 R25.2 R26.2 R27.2 R28.2 R29.2 R30.2 R31.2 R32.2 R33.2 U1.H4 U1.J4
VDD33_C: C12.1 C66.1 JP5.1 JP6.1 LED2.P LED3.P LED4.P LED5.P M3.2 R37.2 R38.2 R39.2 R40.2 R41.2 R42.2 R43.2 R44.2 R45.2 R46.2 R47.2 R48.2 R49.2 R54.2 R117.2 R118.2 R119.2 R120.2 R121.2 U1.A4 U1.B4 U2.5 U3.5
VIN: J1.25 J1.26 J2.25 J2.26 J3.25 J3.26 J7.25 J7.26 J8.25 J8.26 J9.25 J9.26 R1.1 R9.1 R19.1 R34.1 TP9.TP
VIN_A: C1.1 R1.2 U1.R5
VIN_B: C5.1 R19.2 U1.H5
VIN_C: C9.1 R34.2 U1.A5
VIN_EN_A: J1.3 J7.3 R8.1 R109.2 U1.W5
VIN_EN_B: J2.3 J8.3 R25.1 R110.2 U1.L5
VIN_EN_C: J3.3 J9.3 R41.1 R111.2 U1.D5
VIN_SNS_A: J1.4 J7.4 R112.2 U1.T5
VIN_SNS_B: J2.4 J8.4 R113.2 U1.J5
VIN_SNS_C: J3.4 J9.4 R114.2 U1.B5
VIN_SNS_X: J4.P$2 J5.P$2 R112.1 R113.1 R114.1
VSNSM0: C17.1 R58.2 U1.Z5
VSNSM1: C19.1 R60.2 U1.X6
VSNSM2: C21.1 R62.2 U1.Y8
VSNSM3: C23.1 R64.2 U1.X8
VSNSM4: C25.1 R66.2 U1.Y10
VSNSM5: C27.1 R68.2 U1.T9
VSNSM6: C29.1 R70.2 U1.R10
VSNSM7: C31.1 R72.2 U1.T8
VSNSM8: C33.1 R74.2 U1.P5
VSNSM9: C35.1 R76.2 U1.M6
VSNSM10: C37.1 R78.2 U1.N8
VSNSM11: C39.1 R80.2 U1.M8
VSNSM12: C41.1 R82.2 U1.N10
VSNSM13: C43.1 R84.2 U1.J9
VSNSM14: C45.1 R86.2 U1.H10
VSNSM15: C47.1 R88.2 U1.J8
VSNSM16: C49.1 R90.2 U1.G5
VSNSM17: C51.1 R92.2 U1.E6
VSNSM18: C53.1 R94.2 U1.F8
VSNSM19: C55.1 R96.2 U1.E8
VSNSM20: C57.1 R98.2 U1.F10
VSNSM21: C59.1 R100.2 U1.B9
VSNSM22: C61.1 R102.2 U1.A10
VSNSM23: C63.1 R104.2 U1.B8
VSNSM_CH0: J1.46 J7.46 R58.1
VSNSM_CH1: J1.40 J7.40 R60.1
VSNSM_CH2: J1.36 J7.36 R62.1
VSNSM_CH3: J1.34 J7.34 R64.1
VSNSM_CH4: J1.30 J7.30 R66.1
VSNSM_CH5: J1.18 J7.18 R68.1
VSNSM_CH6: J1.16 J7.16 R70.1
VSNSM_CH7: J1.14 J7.14 R72.1
VSNSM_CH8: J2.46 J8.46 R74.1
VSNSM_CH9: J2.40 J8.40 R76.1
VSNSM_CH10: J2.36 J8.36 R78.1
VSNSM_CH11: J2.34 J8.34 R80.1
VSNSM_CH12: J2.30 J8.30 R82.1
VSNSM_CH13: J2.18 J8.18 R84.1
VSNSM_CH14: J2.16 J8.16 R86.1
VSNSM_CH15: J2.14 J8.14 R88.1
VSNSM_CH16: J3.46 J9.46 R90.1
VSNSM_CH17: J3.40 J9.40 R92.1
VSNSM_CH18: J3.36 J9.36 R94.1
VSNSM_CH19: J3.34 J9.34 R96.1
VSNSM_CH20: J3.30 J9.30 R98.1
VSNSM_CH21: J3.18 J9.18 R100.1
VSNSM_CH22: J3.16 J9.16 R102.1
VSNSM_CH23: J3.14 J9.14 R104.1
VSNSP0: C16.1 R57.2 U1.Z4
VSNSP1: C18.1 R59.2 U1.X5
VSNSP2: C20.1 R61.2 U1.Y7
VSNSP3: C22.1 R63.2 U1.X7
VSNSP4: C24.1 R65.2 U1.Y9
VSNSP5: C26.1 R67.2 U1.U9
VSNSP6: C28.1 R69.2 U1.R9
VSNSP7: C30.1 R71.2 U1.R8
VSNSP8: C32.1 R73.2 U1.P4
VSNSP9: C34.1 R75.2 U1.M5
VSNSP10: C36.1 R77.2 U1.N7
VSNSP11: C38.1 R79.2 U1.M7
VSNSP12: C40.1 R81.2 U1.N9
VSNSP13: C42.1 R83.2 U1.K9
VSNSP14: C44.1 R85.2 U1.H9
VSNSP15: C46.1 R87.2 U1.H8
VSNSP16: C48.1 R89.2 U1.G4
VSNSP17: C50.1 R91.2 U1.E5
VSNSP18: C52.1 R93.2 U1.F7
VSNSP19: C54.1 R95.2 U1.E7
VSNSP20: C56.1 R97.2 U1.F9
VSNSP21: C58.1 R99.2 U1.C9
VSNSP22: C60.1 R101.2 U1.A9
VSNSP23: C62.1 R103.2 U1.A8
VSNSP_CH0: J1.45 J7.45 R57.1
VSNSP_CH1: J1.39 J7.39 R59.1
VSNSP_CH2: J1.35 J7.35 R61.1
VSNSP_CH3: J1.33 J7.33 R63.1
VSNSP_CH4: J1.29 J7.29 R65.1
VSNSP_CH5: J1.17 J7.17 R67.1
VSNSP_CH6: J1.15 J7.15 R69.1
VSNSP_CH7: J1.13 J7.13 R71.1
VSNSP_CH8: J2.45 J8.45 R73.1
VSNSP_CH9: J2.39 J8.39 R75.1
VSNSP_CH10: J2.35 J8.35 R77.1
VSNSP_CH11: J2.33 J8.33 R79.1
VSNSP_CH12: J2.29 J8.29 R81.1
VSNSP_CH13: J2.17 J8.17 R83.1
VSNSP_CH14: J2.15 J8.15 R85.1
VSNSP_CH15: J2.13 J8.13 R87.1
VSNSP_CH16: J3.45 J9.45 R89.1
VSNSP_CH17: J3.39 J9.39 R91.1
VSNSP_CH18: J3.35 J9.35 R93.1
VSNSP_CH19: J3.33 J9.33 R95.1
VSNSP_CH20: J3.29 J9.29 R97.1
VSNSP_CH21: J3.17 J9.17 R99.1
VSNSP_CH22: J3.15 J9.15 R101.1
VSNSP_CH23: J3.13 J9.13 R103.1
WP: JP7.1 R56.1 U1.A2 U1.H2 U1.R2

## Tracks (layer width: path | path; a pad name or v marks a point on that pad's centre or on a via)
ALERTB  (via drill 0.2, 0.2 pad 0.23, 0.2 pad 0.25)
  Route2 0.1: v205.8,58 v136.9,58 v130.1,58 v124.1,58 v108.8,58 | J5.P$6 260.35,49.65 | 259.4,50.6 v205.8,50.6 | v12,55.6 v108.8,55.6
  Route2 0.15: 260.35,49.65 259.4,50.6
  Route15 0.1: U1.F2 136.1,54.1 136.5,54.5 136.5,56.3 136.9,56.7 v136.9,58 | v124.1,58 124.1,55.8 124.5,55.4 124.5,54 U1.Y2 | U1.N2 130.1,54 v130.1,58 | TP3.TP 205.74,80.86 205.8,80.8 v205.8,61 v205.8,58 v205.8,50.6 | J4.P$6 7.62,49.62 | v108.8,55.6 v108.8,58
  Route15 0.15: 7.62,49.62 8.8,50.8 11.2,50.8 12,51.6 v12,55.6
  Bottom 0.1: TP3.TP 205.75,81.1 205.75,78.15 R51.1 | v205.8,61 211.31,61 R121.1
  other vias: 136.1,53.6 124.9,53.6 130.5,53.6
  pour Route15 (no thermals): 205.8,78.6 205.7,79.2 205.4,79.7 206.2,79.7 205.9,79.2
  pour Bottom (no thermals): 205.75,78.6 205.65,79 205.3,79.5 206.2,79.5 205.85,79
ASEL0_A  (via drill 0.2, 0.2 pad 0.23)
  Route2 0.1: v123.3,52.8 122.9,52.8 121.6,54.1 120.5,54.1 120.4,54 v57.2,54
  Route15 0.1: U1.Y3 v123.3,52.8 | v57.2,54 57.2,58.2 55.95,59.45 JP2.3 JP2.2
  other vias: 124.9,52.8
ASEL0_B  (via drill 0.2, 0.2 pad 0.25)
  Route2 0.1: v129.7,61 84,61 82.7,62.3 69.43,62.3 JP4.2
  Route15 0.1: JP4.3 JP4.2
  Bottom 0.1: U1.N3 130.1,53.2 130.1,55.4 129.7,55.8 v129.7,61
  other vias: 130.5,52.8
ASEL0_C  (via drill 0.2)
  Top 0.1: U1.F3 136.5,53.2 136.5,57.4 136.4,57.5 136.4,59.1 v136.9,59.6
  Route2 0.1: v136.9,59.6 131.3,59.6 131,59.9 129.5,59.9 129.2,59.6 128.4,59.6 127.8,60.2 83.8,60.2 82.55,61.45 JP6.2
  Route15 0.1: JP6.3 JP6.2
ASEL1_A  (via drill 0.2, 0.2 pad 0.23)
  Route2 0.1: v122.2,59.4 83.8,59.4 82.8,60.4 51.8,60.4 50.85,59.45 JP1.3
  Route15 0.1: U1.X3 125.3,53.2 123,53.2 122.2,54 v122.2,59.4 | JP1.2 JP1.3
  other vias: 125.7,52.8
ASEL1_B  (via drill 0.2, 0.2 pad 0.25)
  Route2 0.1: v130.5,61 130.1,61.4 84.4,61.4 83.2,62.6 64.65,62.6 JP3.2
  Route15 0.1: JP3.3 JP3.2
  Bottom 0.1: U1.M3 130.9,53.2 130.9,55.2 130.5,55.6 v130.5,61
  other vias: 131.3,52.8
ASEL1_C  (via drill 0.2, 0.2 pad 0.25)
  Route2 0.1: v137.7,57.2 136.7,57.2 136.3,57.6 83.1,57.6 82.2,58.5 77.15,58.5 JP5.3
  Route15 0.1: JP5.2 JP5.3
  Bottom 0.1: U1.E3 137.3,53.2 137.3,56.8 v137.7,57.2
  other vias: 136.9,52.8
AUX_SCL  (via drill 0.2)
  Route15 0.15: 25,77 26.59,78.59 J6.11
  Route15 0.152: v11.6,77 25,77 | J6.11 26.59,80.34
  Bottom 0.152: U4.1 8.4,75.71 8.5,76 8.5,76.6 8.9,77 v11.6,77 13.21,77 13.72,77.01 14.9,77.01 R106.1
AUX_SDA  (via drill 0.2)
  Route2 0.152: v11.64,75.69 14.3,78.3 24.5,78.3 25.6,79.4 25.6,81.2 J6.12
  Bottom 0.152: R105.1 13.97,74.68 12.95,75.69 v11.64,75.69 10.38,75.69 U4.3
AUXFAULTB_3V3  (via drill 0.2)
  Top 0.15: R110.1 255.27,46.99 | v253,43.9 253,45.13 R111.1
  Top 0.152: R109.1 R110.1 R111.1 | 255.27,46.99 256.54,48.26 259.08,48.26 J5.P$4
  Route2 0.15: v9.04,6.8 10.84,5 82.2,5 85,7.8 90.2,7.8 93,5 171.1,5 173.9,7.8 179.1,7.8 181.9,5 253.97,5 255.16,6.2 255.16,20.8 253,23.6 v253,43.9
  Route15 0.15: J4.P$4 7.59,46.99 6.2,45.6 6.2,38 9.04,35.16 v9.04,6.8
CTRL0  (via drill 0.2)
  Top 0.1: R35.1 170.5,69.6 170.7,69.8 | 173.36,69.8 S1.5 | R107.1 251.33,52.07 251.2,52 v249.6,52
  Top 0.15: R2.1 R20.1 R35.1 | 170.7,69.8 173.36,69.8
  Route2 0.1: v249.6,52 204.97,52.2 204.56,51.8 203.37,51.8 203.16,52 v178,52
  Route15 0.1: TP14.TP 175.2,80.6 175.2,71.6 S1.2 178,68.76 v178,52
  Bottom 0.1: 171.45,69.85 171.23,69.63 C13.1
  Bottom 0.15: R50.2 S1.2 S1.5 171.45,69.85
  pour Route15 (no thermals): 175.2,78.6 175.1,79.2 174.8,79.7 175.6,79.7 175.3,79.2
CTRL0_A  (via drill 0.2)
  Top 0.1: U1.F1 v136.1,55.2
  Top 0.15: v148.1,65.5 R37.1 | R35.2 v170.4,66.9
  Route2 0.1: v136.9,62.2 v148.1,62.2 v170.4,62.2
  Route15 0.1: v136.1,55.2 136.1,56.3 136.4,56.6 136.4,60 136.9,60.5 v136.9,62.2 | v148.1,62.2 v148.1,65.5 | v170.4,66.9 v170.4,62.2
CTRL0_B  (via drill 0.2)
  Top 0.1: U1.N1 130.5,56.8 v130.9,57.2 | 131.6,66.21 R23.1
  Top 0.15: v131.6,65.4 131.6,66.21 | R20.2 v168.6,66.9
  Route2 0.1: v168.6,64.8 132.2,64.8 v131.6,65.4
  Route15 0.1: v130.9,57.2 130.9,64.7 v131.6,65.4 | v168.6,66.9 v168.6,64.8
CTRL0_C  (via drill 0.2)
  Top 0.1: U1.Y1 v124.9,55.2
  Top 0.15: v112.3,65.5 R6.1 | v166.8,66.9 R2.2
  Route2 0.1: v124.9,55.2 124.2,55.2 123.8,55.6 122.2,55.6 121.9,55.9 v112.3,55.9 | v124.1,62.6 v166.8,62.6
  Route15 0.1: v112.3,55.9 v112.3,65.5 | v124.9,55.2 124.9,55.7 124.6,56 124.6,58.4 124.1,58.9 v124.1,62.6 | v166.8,62.6 v166.8,66.9
CTRL0_X  (via drill 0.2)
  Top 0.152: R107.2 253.17,52.07 253.2,52.1 254.1,52.1 255.3,53.3 259.08,53.3 J5.P$8
  Route2 0.15: v8.23,7.6 8.23,6 9.84,4.4 82.4,4.4 85.2,7.2 90,7.2 92.8,4.4 171.3,4.4 174.1,7.2 178.9,7.2 181.7,4.4 255.37,4.4 257.6,6.6 257.6,38.2 261.6,42.2 261.6,50.82 J5.P$8
  Route15 0.15: J4.P$8 6.07,52.07 5.4,51.4 5.4,37.4 8.23,34.56 v8.23,7.6
CTRL1  (via drill 0.2)
  Top 0.1: R36.1 187.8,69.7 187.7,69.8 | 184.58,69.8 S2.2 | R108.1 251.25,57.15 251.2,57.2 v250.2,57.2
  Top 0.15: R3.1 R21.1 R36.1 | 187.7,69.8 184.58,69.8
  Route2 0.1: v250.2,57.2 249,56 211.2,56 210.8,56.4 v185.6,56.4
  Route15 0.1: TP15.TP 182.8,81 182.8,71.6 S2.2 185.6,68.78 v185.6,56.4
  Bottom 0.1: 186.69,69.85 186.91,69.63 C14.1
  Bottom 0.15: R50.1 S2.5 S2.2 186.69,69.85
  pour Route15 (no thermals): 182.8,78.6 182.7,79.2 182.4,79.7 183.2,79.7 182.9,79.2
CTRL1_A  (via drill 0.2)
  Top 0.15: v149.9,65.5 R38.1 | R36.2 v187.8,66.8
  Route2 0.1: v136.1,60.6 v149.9,60.6 | v187.8,63.7 v149.9,63.7
  Route15 0.1: U1.G3 135.7,53.2 135.7,56.5 136.1,56.9 v136.1,60.6 | v149.9,60.6 v149.9,63.7 | v149.9,63.7 v149.9,65.5 | v187.8,66.8 v187.8,63.7 | v149.9,63.7 149.9,63.5
  other vias: 135.3,52.8
CTRL1_B  (via drill 0.2)
  Top 0.1: U1.P3 129.3,53.2 128.7,53.2 128.5,53.4 128.5,56.8 v128.1,57.2 | 128.1,66.1 128,66.21 R24.1
  Top 0.15: v128.1,65.4 128.1,66.1 | R21.2 v189.6,66.8
  Route2 0.1: v189.6,64.4 187,64.4 186.8,64.2 129.3,64.2 v128.1,65.4
  Route15 0.1: v128.1,57.2 v128.1,65.4 | v189.6,66.8 v189.6,64.4
  other vias: 129.7,52.8
CTRL1_C  (via drill 0.2)
  Top 0.1: U1.Z3 v123.3,53.6
  Top 0.15: v110.5,65.5 R7.1 | R3.2 v191.4,63.2
  Route2 0.1: v191.4,63.2 150.4,63.2 150.2,63 149.6,63 149.4,63.2 147,63.2 146.8,63 145.8,63 145.6,63.2 v110.5,63.2 | v123.3,53.6 122.8,53.6 121.9,54.5 v110.5,54.5
  Route15 0.1: v110.5,65.5 v110.5,63.2 v110.5,54.5
CTRL1_X  (via drill 0.2)
  Top 0.152: J5.P$12 259.1,58.4 256.4,58.4 255.2,57.2 253.4,57.2 253.35,57.15 R108.2
  Route2 0.1: v251,58.4 259.1,58.4 260.3,57.2 260.3,57.13 260.26,57.17 260.27,57.17 J5.P$12 | v251,70.8 171.8,70.8 171.2,71.4 113.8,71.4 113.4,71 v34.2,71
  Route2 0.15: v34.2,59.4 12,59.4 11,58.4 8.77,58.4 J4.P$12
  Route15 0.1: v251,58.4 v251,70.8 | v34.2,71 v34.2,59.4
CTRL2  (via drill 0.2)
  Route2 0.1: 254.59,54.61 254.4,54.8 v248.8,54.8 | v248.8,68.2 185.4,68.2 185.2,68.4 172.4,68.4 170.4,70.4 114.8,70.4 114.2,69.8 v36.2,69.8 | 10.55,55 J4.P$9
  Route2 0.15: J5.P$9 254.59,54.61 | v36.2,55 10.55,55
  Route15 0.1: v248.8,54.8 v248.8,68.2 | v36.2,69.8 v36.2,55
CTRL3  (via drill 0.2)
  Route2 0.1: J5.P$10 260.35,54.55 | 259.2,53.4 255.8,53.4 255,54.2 v248.2,54.2 | v248.2,68.8 173,68.8 171,70.8 114.2,70.8 113.8,70.4 v36.8,70.4
  Route2 0.15: 260.35,54.55 259.2,53.4 | v36.8,54.4 12.4,54.4 11.4,53.4 8.83,53.4 J4.P$10
  Route15 0.1: v248.2,54.2 v248.2,68.8 | v36.8,70.4 v36.8,54.4
DACM_CH0
  Top 0.152: J1.43 24.77,11.43 24.77,17.78 J7.43
DACM_CH1
  Bottom 0.152: J1.42 24.77,8.89 24.77,15.24 J7.42
DACM_CH2
  Bottom 0.152: J1.38 29.84,8.89 29.84,15.24 J7.38
DACM_CH3
  Bottom 0.152: J1.32 37.47,8.89 37.47,15.24 J7.32
DACM_CH4
  Top 0.152: J1.27 45.09,11.43 45.09,17.78 J7.27
DACM_CH5
  Bottom 0.152: J1.24 47.62,8.89 47.62,15.24 J7.24
DACM_CH6
  Top 0.152: J1.21 52.7,11.43 52.7,17.78 J7.21
DACM_CH7
  Bottom 0.152: J1.20 52.7,8.89 52.7,15.24 J7.20
DACM_CH8
  Top 0.152: J2.43 113.03,11.43 113.03,17.78 J8.43
DACM_CH9
  Bottom 0.152: J2.42 113.03,8.89 113.03,15.24 J8.42
DACM_CH10
  Bottom 0.152: J2.38 118.11,8.89 118.11,15.24 J8.38
DACM_CH11
  Bottom 0.152: J2.32 125.73,8.89 125.73,15.24 J8.32
DACM_CH12
  Top 0.152: J2.27 133.35,11.43 133.35,17.78 J8.27
DACM_CH13
  Bottom 0.152: J2.24 135.89,8.89 135.89,15.24 J8.24
DACM_CH14
  Top 0.152: J2.21 140.97,11.43 140.97,17.78 J8.21
DACM_CH15
  Bottom 0.152: J2.20 140.97,8.89 140.97,15.24 J8.20
DACM_CH16
  Top 0.152: J3.43 201.29,11.43 201.29,17.78 J9.43
DACM_CH17
  Bottom 0.152: J3.42 201.29,8.89 201.29,15.24 J9.42
DACM_CH18
  Bottom 0.152: J3.38 206.38,8.89 206.38,15.24 J9.38
DACM_CH19
  Bottom 0.152: J3.32 214,8.89 214,15.24 J9.32
DACM_CH20
  Top 0.152: J3.27 221.62,11.43 221.62,17.78 J9.27
DACM_CH21
  Bottom 0.152: J3.24 224.16,8.89 224.16,15.24 J9.24
DACM_CH22
  Top 0.152: J3.21 229.24,11.43 229.24,17.78 J9.21
DACM_CH23
  Bottom 0.152: J3.20 229.24,8.89 229.24,15.24 J9.20
DACP_CH0  (via drill 0.2, 0.2 pad 0.23)
  Route2 0.1: U1.Y4 124.5,52.4 122.8,52.4 122,53.2 v23.64,53.2
  Route15 0.1: v23.64,53.2 23.64,21 22.43,19.8 22.43,17.57 J7.44
  Bottom 0.152: J1.44 22.23,8.89 22.23,15.24 J7.44
  other vias: 124.9,52
DACP_CH1  (via drill 0.2, 0.2 pad 0.25)
  Top 0.152: J1.41 27.3,11.43 27.3,17.78 J7.41
  Route2 0.1: U1.Y6 123.3,50.4 122.1,51.6 30.2,51.6 30,51.8 v26.04,51.8
  Route15 0.1: v26.04,51.8 J7.41
  other vias: 124.9,50.4
DACP_CH2  (via drill 0.2)
  Top 0.1: U1.Z7 v123.3,49.6
  Top 0.152: J1.37 32.38,11.43 32.38,17.78 J7.37
  Route2 0.1: v123.3,49.6 v31.14,49.6
  Route15 0.1: v31.14,49.6 31.14,19.07 J7.37
DACP_CH3  (via drill 0.2)
  Top 0.152: J1.31 40.01,11.43 40.01,17.78 J7.31
  Route2 0.1: v124,39.8 v38.73,39.8
  Route15 0.1: v38.73,39.8 J7.31 | U1.Z10 124.1,42 124,41.9 v124,39.8
  other vias: 124.1,47.2
DACP_CH4  (via drill 0.2)
  Route2 0.1: v125.2,41 v43.8,41
  Route15 0.1: v43.8,41 43.8,20.8 42.8,19.8 42.8,17.49 J7.28 | U1.X10 125.7,42.8 125.2,42.3 v125.2,41
  Bottom 0.152: J1.28 42.55,8.89 42.55,15.24 J7.28
  other vias: 125.7,47.2
DACP_CH5  (via drill 0.2, 0.2 pad 0.25)
  Top 0.152: J1.23 50.16,11.43 50.16,17.78 J7.23
  Route2 0.1: v125.8,41.6 v48.9,41.6
  Route15 0.1: v48.9,41.6 48.9,19.09 J7.23 | U1.W9 126.1,47.6 126.1,42.6 125.8,42.3 v125.8,41.6
  other vias: 126.5,48
DACP_CH6  (via drill 0.2)
  Route2 0.1: v125.3,44 125,44 124.8,43.8 58.1,43.8 57.9,44 57.1,44 56.9,43.8 v51.4,43.8
  Route15 0.1: v51.4,43.8 51.4,20.8 50.4,19.8 50.4,17.51 J7.22 | U1.W8 125.3,47.6 v125.3,44
  Bottom 0.152: J1.22 50.16,8.89 50.16,15.24 J7.22
  other vias: 126.5,48.8
DACP_CH7  (via drill 0.2, 0.2 pad 0.23)
  Top 0.152: J1.19 55.24,11.43 55.24,17.78 J7.19
  Route2 0.1: U1.U8 126.9,48.4 126.2,48.4 125.3,47.5 125.3,44.9 124.6,44.2 58.3,44.2 58.1,44.4 v54,44.4
  Route15 0.1: v54,44.4 54,19.11 J7.19
  other vias: 127.3,48.8
DACP_CH8  (via drill 0.2, 0.2 pad 0.25)
  Route2 0.1: U1.N4 130.1,52.4 127.7,52.4 125.7,54.4 123.3,54.4 122.9,54.8 121.8,54.8 121.6,55 v112.2,55
  Route15 0.1: v112.2,55 112.2,21.2 110.8,19.8 110.8,17.47 J8.44
  Bottom 0.152: J2.44 110.49,8.89 110.49,15.24 J8.44
  other vias: 130.5,52
DACP_CH9  (via drill 0.2, 0.2 pad 0.25)
  Top 0.15: v114.3,22 J8.41
  Top 0.152: J2.41 115.57,11.43 115.57,17.78 J8.41
  Route2 0.1: v129.7,22 v114.3,22
  Route15 0.1: v129.7,46.4 v129.7,22
  Bottom 0.1: U1.N6 130.1,50 130.1,46.8 v129.7,46.4
  other vias: 130.5,50.4
DACP_CH10  (via drill 0.2, 0.2 pad 0.25)
  Top 0.152: J2.37 120.65,11.43 120.65,17.78 J8.37
  Route2 0.1: v127.4,20.4 120.73,20.4 J8.37
  Route15 0.1: v127.7,44.8 127.7,20.7 v127.4,20.4
  Bottom 0.1: U1.P7 129.3,49.2 129.3,47 129.1,46.8 128.6,46.8 127.7,45.9 v127.7,44.8
  other vias: 129.7,49.6
DACP_CH11  (via drill 0.2)
  Top 0.152: J2.31 128.27,11.43 128.27,17.78 J8.31
  Route15 0.1: v128.1,45.6 128.1,20.15 J8.31
  Bottom 0.1: U1.P10 129.7,46.8 129.5,46.8 128.8,46.1 128.6,46.1 v128.1,45.6
  other vias: 129.7,47.2
DACP_CH12  (via drill 0.2)
  Top 0.1: U1.M10 v132.1,46.4
  Route15 0.1: v132.1,46.4 132.1,20.8 131.1,19.8 131.1,17.49 J8.28
  Bottom 0.152: J2.28 130.81,8.89 130.81,15.24 J8.28
DACP_CH13  (via drill 0.2, 0.2 pad 0.25)
  Top 0.152: J2.23 138.43,11.43 138.43,17.78 J8.23
  Route2 0.1: U1.L9 132.5,47.6 132.5,46.1 132.6,46 132.8,45.9 132.9,45.7 132.9,44.4 v133.3,44
  Route15 0.1: v133.3,44 133.3,31.9 134.8,30.4 134.8,21.41 J8.23
  other vias: 132.1,48
DACP_CH14  (via drill 0.2 pad 0.25)
  Route15 0.1: U1.L8 132.5,48.4 132.5,46.2 133.2,45.6 133.2,44.7 133.7,44.2 133.7,32.2 135.2,30.7 135.2,21.8 136.8,20.2 137.6,20.2 138.3,19.5 138.3,17.91 J8.22
  Bottom 0.152: J2.22 138.43,8.89 138.43,15.24 J8.22
  other vias: 132.1,48.8
DACP_CH15  (via drill 0.2, 0.2 pad 0.25)
  Top 0.152: J2.19 143.51,11.43 143.51,17.78 J8.19
  Route2 0.1: U1.K8 133.3,48.4 133.3,47.6 133.7,47.2 v133.7,46.4
  Route15 0.1: v133.7,46.4 133.7,46 134.9,44.8 134.9,34.1 138.2,30.8 138.2,21.2 139.2,20.2 141.09,20.2 J8.19
  other vias: 132.9,48.8
DACP_CH16  (via drill 0.2, 0.2 pad 0.25)
  Route2 0.1: U1.F4 136.5,52.4 137.2,52.4 137.6,52.8 139.8,52.8 140.4,53.4 140.4,53.7 141,54.3 v198.97,54.3
  Route15 0.1: v198.97,54.3 198.97,17.57 J9.44
  Bottom 0.152: J3.44 198.75,8.89 198.75,15.24 J9.44
  other vias: 136.1,52
DACP_CH17  (via drill 0.2)
  Top 0.152: J3.41 203.84,11.43 203.84,17.78 J9.41
  Route2 0.1: v146.2,34.2 v202.6,34.2
  Route15 0.1: v145.4,48 145.4,47.8 146.2,47 v146.2,34.2 | v202.6,34.2 J9.41
  Bottom 0.1: U1.F6 136.5,50.8 142.6,50.8 v145.4,48
  other vias: 136.1,50.4
DACP_CH18  (via drill 0.2)
  Top 0.152: J3.37 208.91,11.43 208.91,17.78 J9.37
  Route2 0.1: v145.8,35.9 v207.6,35.9
  Route15 0.1: v144.6,48 145.8,46.8 v145.8,35.9 | v207.6,35.9 207.6,19.07 J9.37
  Bottom 0.1: U1.G7 135.7,50 142.6,50 v144.6,48
  other vias: 135.3,49.6
DACP_CH19  (via drill 0.2)
  Top 0.1: U1.G10 v135.3,46.4
  Top 0.152: J3.31 216.53,11.43 216.53,17.78 J9.31
  Route2 0.1: v138.1,38.2 v215.2,38.2
  Route15 0.1: v135.3,46.4 135.3,45.8 136.5,44.6 137,44.6 137.3,44.3 137.3,43.4 138.1,42.6 v138.1,38.2 | v215.2,38.2 215.2,19.15 J9.31
DACP_CH20  (via drill 0.2)
  Top 0.1: U1.E10 v136.9,46.4
  Route2 0.1: v140.5,40 v220.37,40
  Route15 0.1: v136.9,46.4 136.9,46 137.2,45.7 138.4,45.7 139.2,44.9 140,44.9 140.5,44.4 v140.5,40 | v220.37,40 220.37,20.8 219.37,19.8 219.37,17.49 J9.28
  Bottom 0.152: J3.28 219.07,8.89 219.07,15.24 J9.28
DACP_CH21  (via drill 0.2)
  Top 0.152: J3.23 226.69,11.43 226.69,17.78 J9.23
  Route2 0.1: v141.6,43 v225.4,43
  Route15 0.1: v137.7,46.4 138.4,46.4 139.4,45.4 140.6,45.4 141.6,44.4 v141.6,43 | v225.4,43 225.4,19.11 J9.23
  Bottom 0.1: U1.D9 137.3,47.6 137.3,46.8 v137.7,46.4
  other vias: 137.7,48
DACP_CH22  (via drill 0.2)
  Route2 0.1: v143.2,43.6 v227.6,43.6
  Route15 0.1: U1.D8 138,48.8 138.3,48.4 140.4,48.4 141.2,47.6 141.2,47 143.2,45 v143.2,43.6 | v227.6,43.6 227.6,20.4 226.97,19.8 226.97,17.51 J9.22
  Bottom 0.152: J3.22 226.69,8.89 226.69,15.24 J9.22
  other vias: 137.7,48.8
DACP_CH23  (via drill 0.2)
  Top 0.152: J3.19 231.78,11.43 231.78,17.78 J9.19
  Route2 0.1: v144,44.2 v230.4,44.2
  Route15 0.1: v142.2,47.2 144,45.4 v144,44.2 | v230.4,44.2 230.4,19.19 J9.19
  Bottom 0.1: U1.C8 138.9,48.4 141,48.4 v142.2,47.2
  other vias: 138.5,48.8
FAULT1  (via drill 0.2)
  Route2 0.1: v254.5,66.4 256.6,66.4 257,66 259.1,66 260.2,64.9 260.28,64.8 J5.P$18 | v254.5,77.6 135.8,77.6 135.2,77 129.2,77 128.6,77.6 102.6,77.6 100.6,79.6 97.6,79.6 95.4,77.4 63.8,77.4 59.8,73.4 v31,73.4
  Route2 0.15: v31,65.8 8.65,65.8 J4.P$18
  Route15 0.1: v254.5,66.4 v254.5,77.6 | v31,73.4 v31,65.8
  Bottom 0.1: R122.1 255.3,64.8 256.5,66 259.1,66 260.2,64.9
  Bottom 0.152: R122.1 255.27,64.8 256.54,66.04 259.08,66.04 J5.P$18
FAULT2  (via drill 0.2)
  Route2 0.1: v253.8,63.5 259.1,63.5 260.3,62.3 260.3,62.2 260.32,62.2 J5.P$16 | v253.8,76.4 103.8,76.4 103,77.2 96,77.2 95.6,76.8 64,76.8 60,72.8 v31.6,72.8
  Route2 0.15: v31.6,63.4 8.79,63.4 J4.P$16
  Route15 0.1: v253.8,63.5 v253.8,76.4 | v31.6,72.8 v31.6,63.4
  Bottom 0.1: 256.6,63.5 259.1,63.5 260.3,62.3
  Bottom 0.152: R123.1 255.3,62.2 256.6,63.5 259.08,63.5 J5.P$16
FAULT3  (via drill 0.2)
  Top 0.152: J5.P$17 257.63,64.77 257.6,64.8 R124.1
  Route2 0.1: 32.37,64.77 v32.4,64.8 | v32.4,72.2 102.8,72.2 104.6,74 v255.4,74
  Route2 0.15: J4.P$17 32.37,64.77
  Route15 0.1: v32.4,64.8 v32.4,72.2 | v255.4,74 255.4,64.8 257.6,64.8 257.63,64.77 J5.P$17
FAULT4  (via drill 0.2)
  Top 0.1: R125.1 257.8,62.2 J5.P$15
  Top 0.152: J5.P$15 257.43,62.23 257.4,62.2 R125.1
  Route2 0.1: v253,63.2 254,62.2 257.8,62.2 J5.P$15 | v253,72.4 186.6,72.4 185.5,73.5 104.7,73.5 102.8,71.6 v33.2,71.6 | 10.19,62.2 J4.P$15
  Route2 0.15: v33.2,62.2 10.19,62.2
  Route15 0.1: v253,63.2 v253,72.4 | v33.2,71.6 v33.2,62.2
FAULTB00  (via drill 0.2)
  Top 0.1: U1.U1 v127.3,55.2 | v138.5,55.2 U1.C1 | U1.K1 v132.9,55.2
  Route2 0.1: v127.3,58.4 v132.9,58.4 v138.5,58.4 210.9,58.4 TP10.1 | v213.4,65.8 v251.8,65.8
  Route15 0.1: TP10.1 213.4,58.5 v213.4,65.8 v213.4,69.6 213.4,80.6 213.36,80.64 TP4.TP | v127.3,55.2 v127.3,58.4 | v138.5,58.4 v138.5,55.2 | v132.9,55.2 v132.9,58.4
  Bottom 0.1: R120.1 R115.2 213,58.1 TP10.1 | U2.2 213.36,70.66 213.3,70.6 213.3,70.5 213.4,70.4 | v251.8,65.8 251.8,64.93 R122.2
  Bottom 0.15: 213.4,70.4 v213.4,69.6
  pour Route15 (no thermals): 213.4,78.6 213.3,79.2 213,79.7 213.8,79.7 213.5,79.2
FAULTB01  (via drill 0.2, 0.2 pad 0.23, 0.2 pad 0.25)
  Top 0.1: U1.U2 126.9,54 126.9,57.3 126.1,58.1 v126.1,58.8 | U1.K2 133.3,54 133.3,57.2 133.7,57.6 v133.7,58.8
  Route2 0.1: v126.1,58.8 v133.7,58.8 v139.3,58.8 213,58.8 TP11.1 215.4,56.4 248.6,56.4 v249.4,57.2
  Route15 0.1: v214.3,69.6 214.3,57.48 TP11.1 | U1.C2 138.5,54.1 138.9,54.5 138.9,56.8 139.3,57.2 v139.3,58.8 | v249.4,57.2 v249.4,61.2
  Bottom 0.1: R119.1 214.8,59.2 | 214.8,59.2 R115.1 214.63,58.97 214.63,58.63 | U2.1 214.31,70.41 214.3,70.4 | 214.63,58.63 214.6,58.6 TP11.1 | 214.8,59.2 214.8,58.8 214.63,58.63 | v249.4,61.2 251.4,61.2 251.8,61.5 251.8,62.07 R123.2
  Bottom 0.15: 214.3,70.4 v214.3,69.6
  other vias: 132.9,53.6 138.5,53.6 127.3,53.6
FAULTB10  (via drill 0.2)
  Top 0.1: U1.W1 v126.5,55.2 | v132.1,55.2 U1.L1 | U1.D1 v137.7,55.2 | R124.2 v250.2,64.8
  Route2 0.1: v126.5,62.2 v132.1,62.2 136,62.2 136.4,61.8 v137.7,61.8 147.6,61.8 147.8,61.6 148.4,61.6 148.6,61.8 218.3,61.8 v218.7,61.4 | v250.2,64.8 v221,64.8
  Route15 0.1: TP5.TP 221,79.46 v221,69.6 v221,64.8 221,58.44 TP12.1 | v126.5,55.2 v126.5,62.2 | v132.1,62.2 132.1,57.8 131.7,57.4 131.7,56.9 132.1,56.5 v132.1,55.2 | v137.7,55.2 137.7,56.2 137.3,56.6 137.3,57.6 137.7,58 v137.7,61.8
  Bottom 0.1: U3.2 220.98,70.58 221,70.5 | TP12.1 219.71,57.21 219.7,57.5 219.7,58.7 R116.2 219.8,59.2 R118.1 219.5,61.4 v218.7,61.4
  Bottom 0.15: 221,70.5 v221,69.6
  pour Route15 (no thermals): 221,78.6 220.9,79.2 220.6,79.7 221.4,79.7 221.1,79.2
FAULTB11  (via drill 0.2, 0.2 pad 0.25)
  Top 0.1: U1.W2 126.1,54 126.1,57 124.9,58.2 v124.9,58.8 | R125.2 v250.2,62.2
  Route2 0.1: v124.9,58.8 125.4,59.3 129.5,59.3 129.8,59.6 130.5,59.6 130.9,59.2 v131.3,59.2 v138.5,59.2 220.1,59.2 TP13.1 | v250.2,62.2 223.6,62.2 v222.8,61.4
  Route15 0.1: v221.9,69.6 221.9,57.5 TP13.1 | v138.5,59.2 138.1,58.8 138.1,54.5 137.7,54.1 U1.D2 | U1.L2 132.1,54.1 131.7,54.5 131.7,56.2 131.3,56.6 v131.3,59.2
  Bottom 0.1: U3.1 221.93,70.43 221.9,70.4 | TP13.1 221.5,57.9 R116.1 221.7,59.1 221.6,59.1 R117.1 221.7,61.2 221.8,61.2 222,61.4 v222.8,61.4
  Bottom 0.15: 221.9,70.4 v221.9,69.6
  other vias: 137.7,53.6 132.1,53.6
FAULTBZ0  (via drill 0.2)
  Route15 0.1: v211.6,73.1 211.6,76.3 v212.2,77
  Bottom 0.1: 213.29,77.85 R52.2
  Bottom 0.15: v212.2,77 212.2,77.57 212.47,77.85 213.29,77.85 | v211.6,73.1 212.39,73.1 U2.4
FAULTBZ1  (via drill 0.2)
  Route15 0.1: v219.8,77 219.2,76.4 v219.2,73.1
  Bottom 0.1: R53.2 220.83,78.07 220.8,77.85 | 220.01,73.1 U3.4
  Bottom 0.15: 220.8,77.85 220.07,77.85 219.8,77.57 v219.8,77 | v219.2,73.1 220.01,73.1
GND  (via drill 0.2 pad 0.25)
  Top 0.1: U1.U3 U1.W3 | U1.W4 U1.U4 | U1.D4 U1.D3 | U1.D4 U1.C4 | U1.G9 U1.G8 135.7,49.2 135.7,50 U1.G6 U1.F5 U1.E4 U1.D4 | U1.L4 U1.K4 | U1.L3 132.5,52.8 | 132.5,52.8 U1.K3 | U1.L3 U1.L4 | U1.L4 U1.M4 U1.N5 U1.P6 129.8,50.4 129.8,50.3 130.1,50 130.1,49.2 U1.P8 U1.P9 129.3,47.6 128.5,47.6 U1.T10 U1.U10 U1.W10 U1.X9 | 133.3,47.2 U1.K10 U1.L10 U1.M9 | 133.3,47.2 U1.J10 | U1.E9 U1.D10 U1.C10 U1.B10 | v138.1,52.4 U1.C4 | U1.C3 U1.C4 | U1.D4 v138.1,52.4 | v138.1,52.4 U1.D3 | U1.D3 138.1,52.8 | 138.1,52.8 U1.C3 | U1.C3 v138.1,52.4 | v132.5,52.4 U1.K3 | U1.K3 U1.K4 | U1.K4 v132.5,52.4 | v132.5,52.4 U1.L4 | v132.5,52.4 U1.L3 | v126.9,52.4 U1.U3 | U1.U4 v126.9,52.4 | U1.W4 U1.W3 | U1.W3 v126.9,52.4 | v126.9,52.4 U1.W4 | U1.W4 U1.X4 U1.Y5 U1.Z6 124.1,50.3 124.5,49.9 124.5,49.2 U1.Z8 U1.Z9 | U1.U3 U1.U4 | U1.U3 127.7,53.2 127.7,55.6 | 124.5,54 124.5,53.4 124.7,53.2 126.1,53.2 U1.W3 | 133.3,47.2 133.3,46 | 132.5,52.8 132.5,55.6 | 138.1,52.8 138.1,55.6
  Bottom 0.1: 135.7,46 135.7,46.8 136.5,46.8 136.5,46 | 133.3,55.6 133.3,54.6 | 131.7,55.6 131.7,54.6 132.5,54.6 | 132.5,54.6 132.5,55.6 | 133.3,54.6 132.5,54.6 | 133.3,54.6 134.1,54.6 134.1,55.6
  other vias: 137.7,47.2 132.1,47.2 126.5,47.2
  pour Bottom (rank 2): 1.27,2.54 1.27,83.82 2.54,85.09 261.62,85.09 262.89,83.82 262.89,2.54 261.62,1.27 2.54,1.27
  pour Top (rank 2): 1.02,2.03 1.02,84.33 2.03,85.34 262.13,85.34 263.14,84.33 263.14,2.03 262.13,1.02 2.03,1.02
  pour Route2 (rank 2): 1,1 263.2,1 263.2,85.4 1,85.4
  pour Route15 (rank 2): 1.2,85.2 263,85.2 263,1.2 1.2,1.2
N$2  (via drill 0.2)
  Top 0.1: v164.3,76.8 162.9,76.8 162.7,77 161.06,77 LED2.N
  Bottom 0.1: R55.1 v164.3,76.8
N$4  (via drill 0.2)
  Top 0.1: v132.1,57.2 132.1,57.23 132.11,57.23 v132.1,57.2
  Top 0.15: LED1.P 132.1,57.23
  Bottom 0.1: v132.1,57.2 132.09,57.89 R22.1
N$8
  Bottom 0.1: M4.3 168.2,74.85 168.2,74.8 167.2,74.8 166.9,74.5 163.8,74.5 163.3,75 163.3,75.52 R55.2
N$28  (via drill 0.2)
  Top 0.1: LED5.N 220.96,77
  Top 0.15: 220.96,77 v221.9,77
  Bottom 0.1: R53.1 221.11,76.2 221.11,76.19 221.2,76.1
  Bottom 0.15: 221.2,76.1 221.7,76.1 221.9,76.3 v221.9,77
N$29  (via drill 0.2)
  Top 0.1: 213.36,77 LED4.N
  Top 0.15: v214.3,77 213.36,77
  Bottom 0.1: 213.42,76.1 R52.1
  Bottom 0.15: v214.3,77 214.3,76.3 214.1,76.1 213.42,76.1
N$30  (via drill 0.2)
  Top 0.1: LED3.N 205.74,76.87 205.61,77
  Top 0.15: 205.61,77 v204.8,77
  Bottom 0.1: 205.68,76.1 R51.2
